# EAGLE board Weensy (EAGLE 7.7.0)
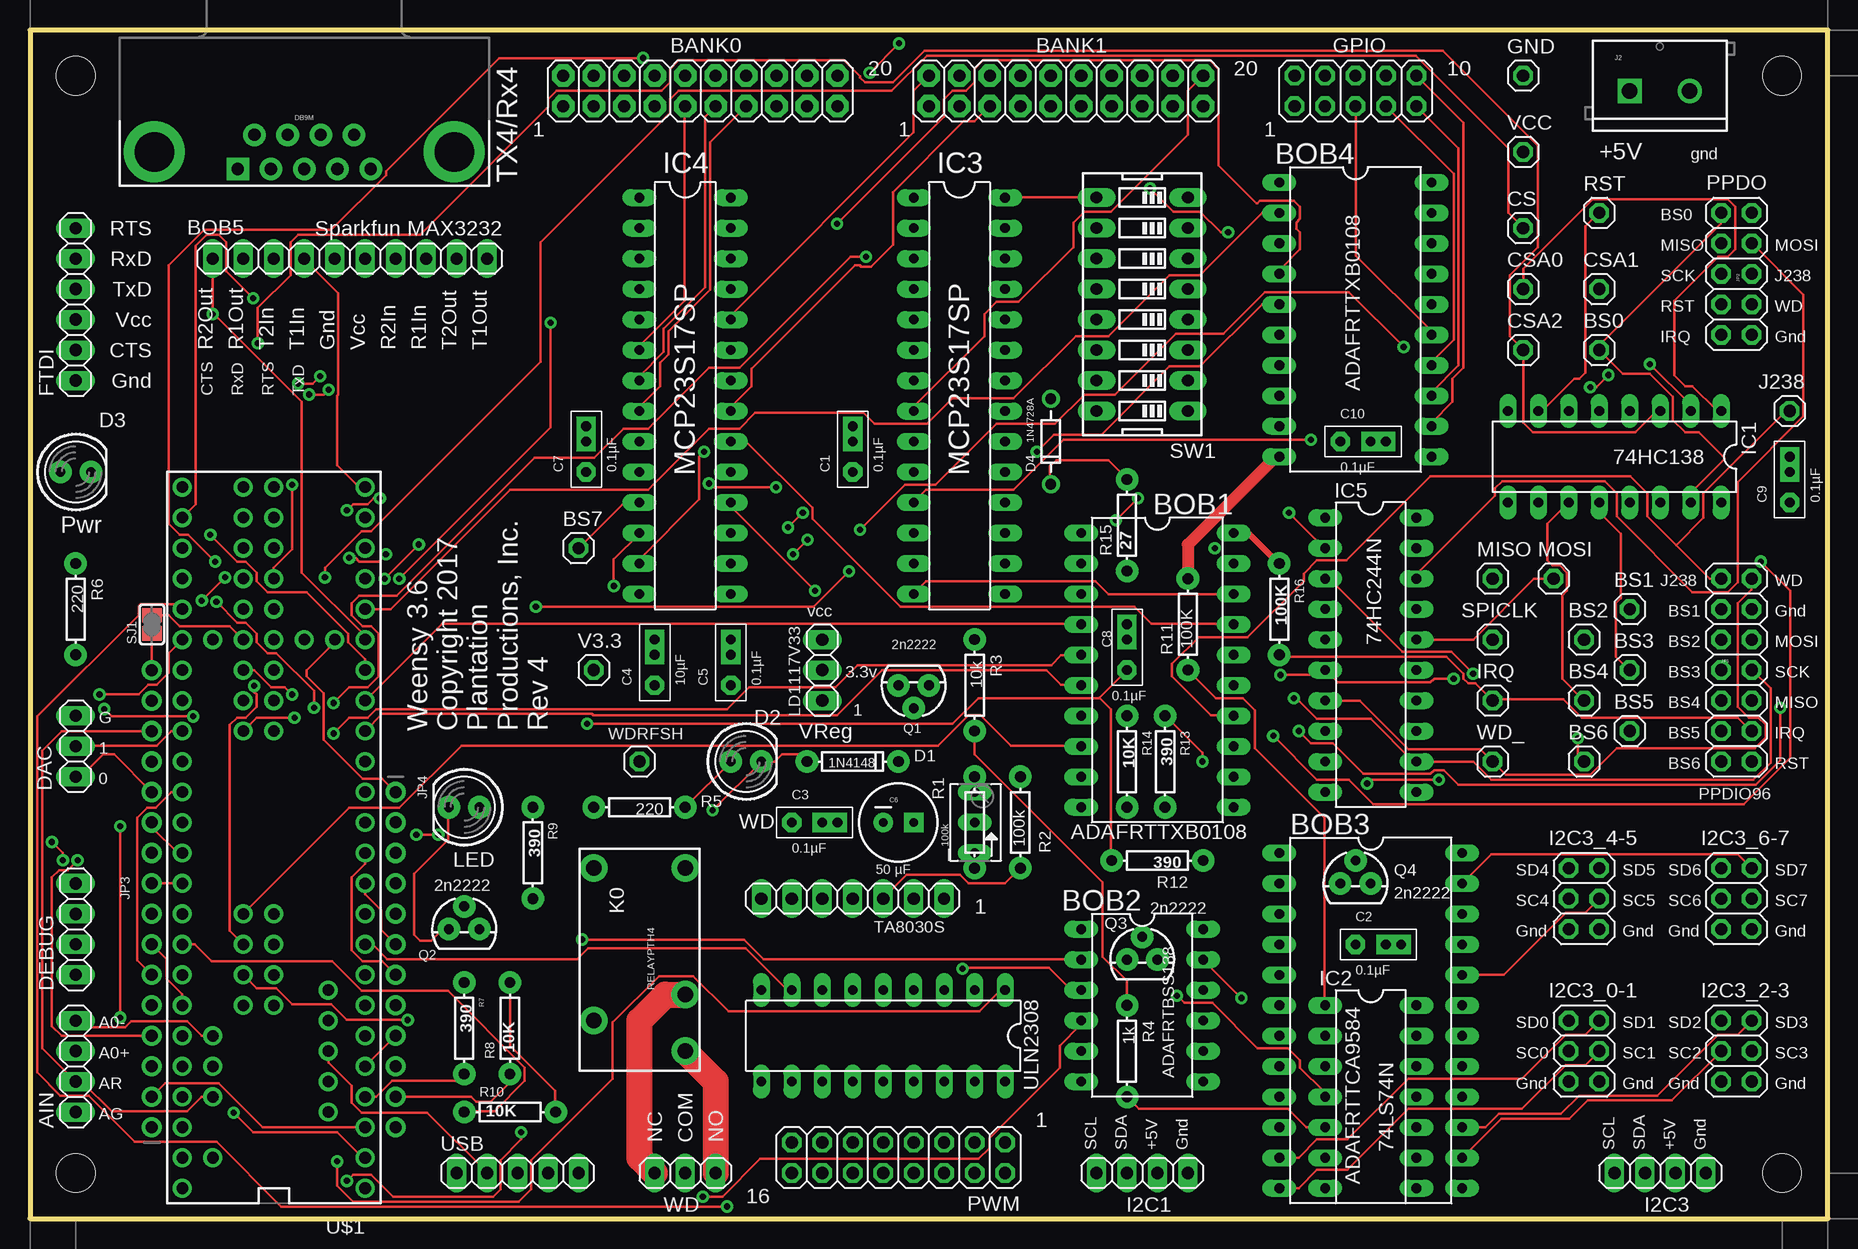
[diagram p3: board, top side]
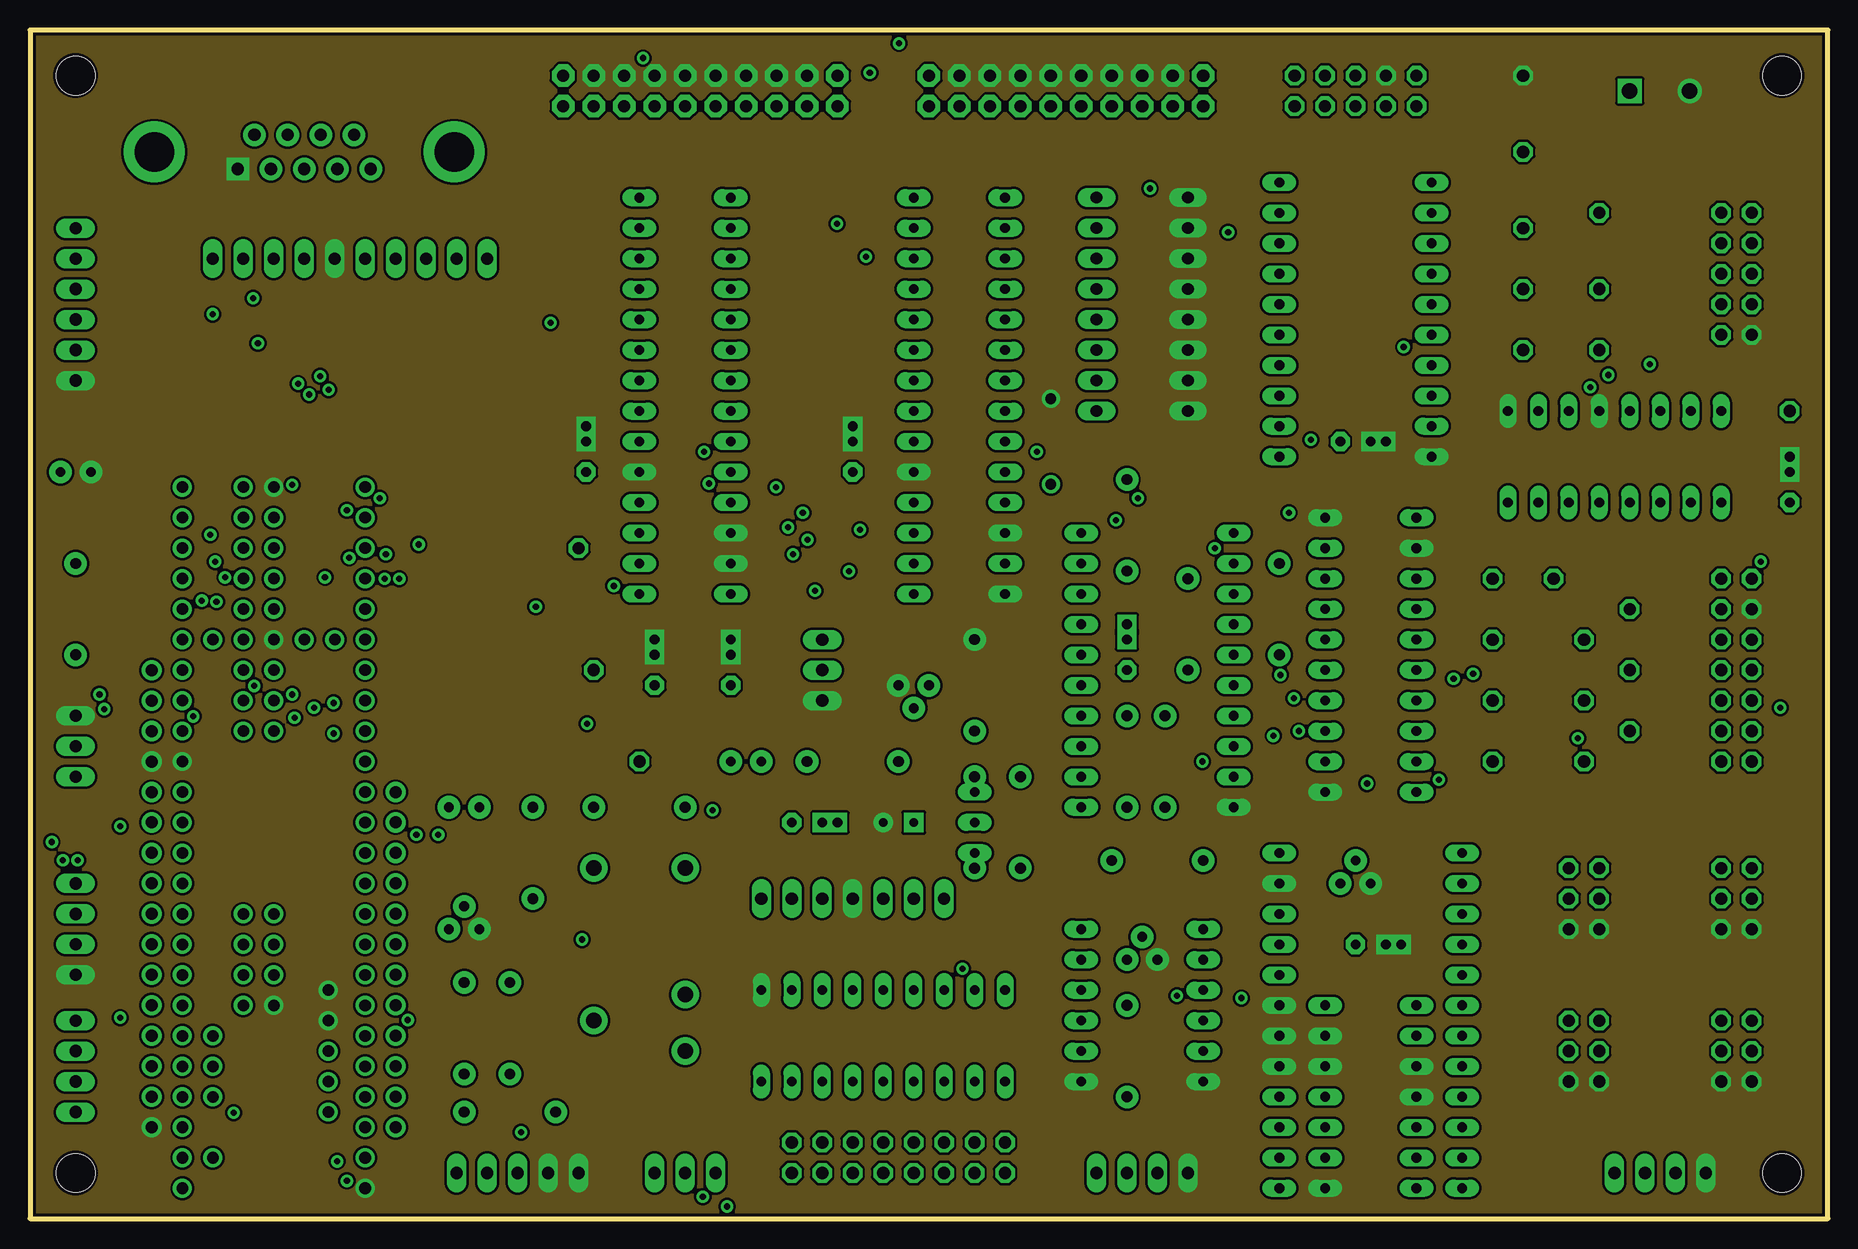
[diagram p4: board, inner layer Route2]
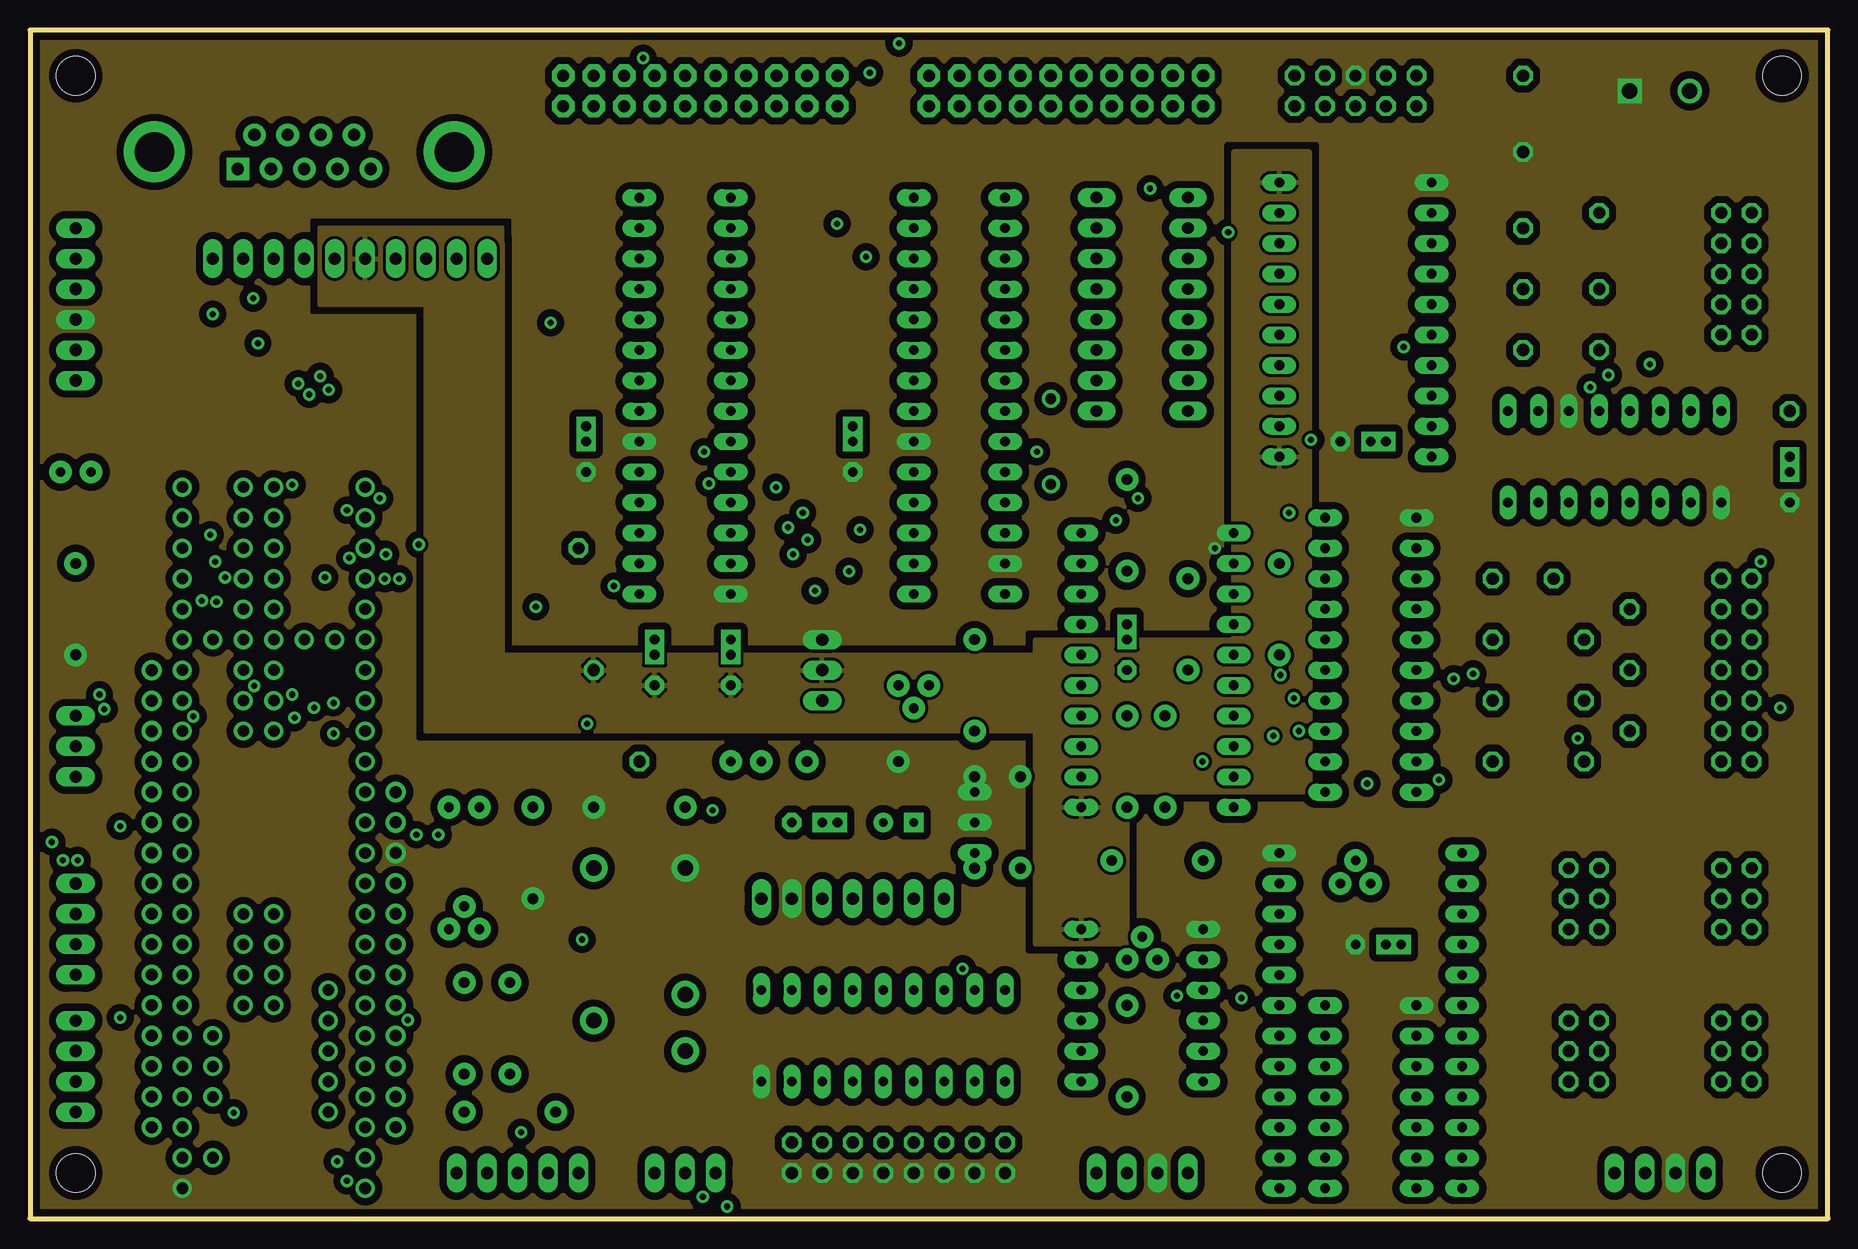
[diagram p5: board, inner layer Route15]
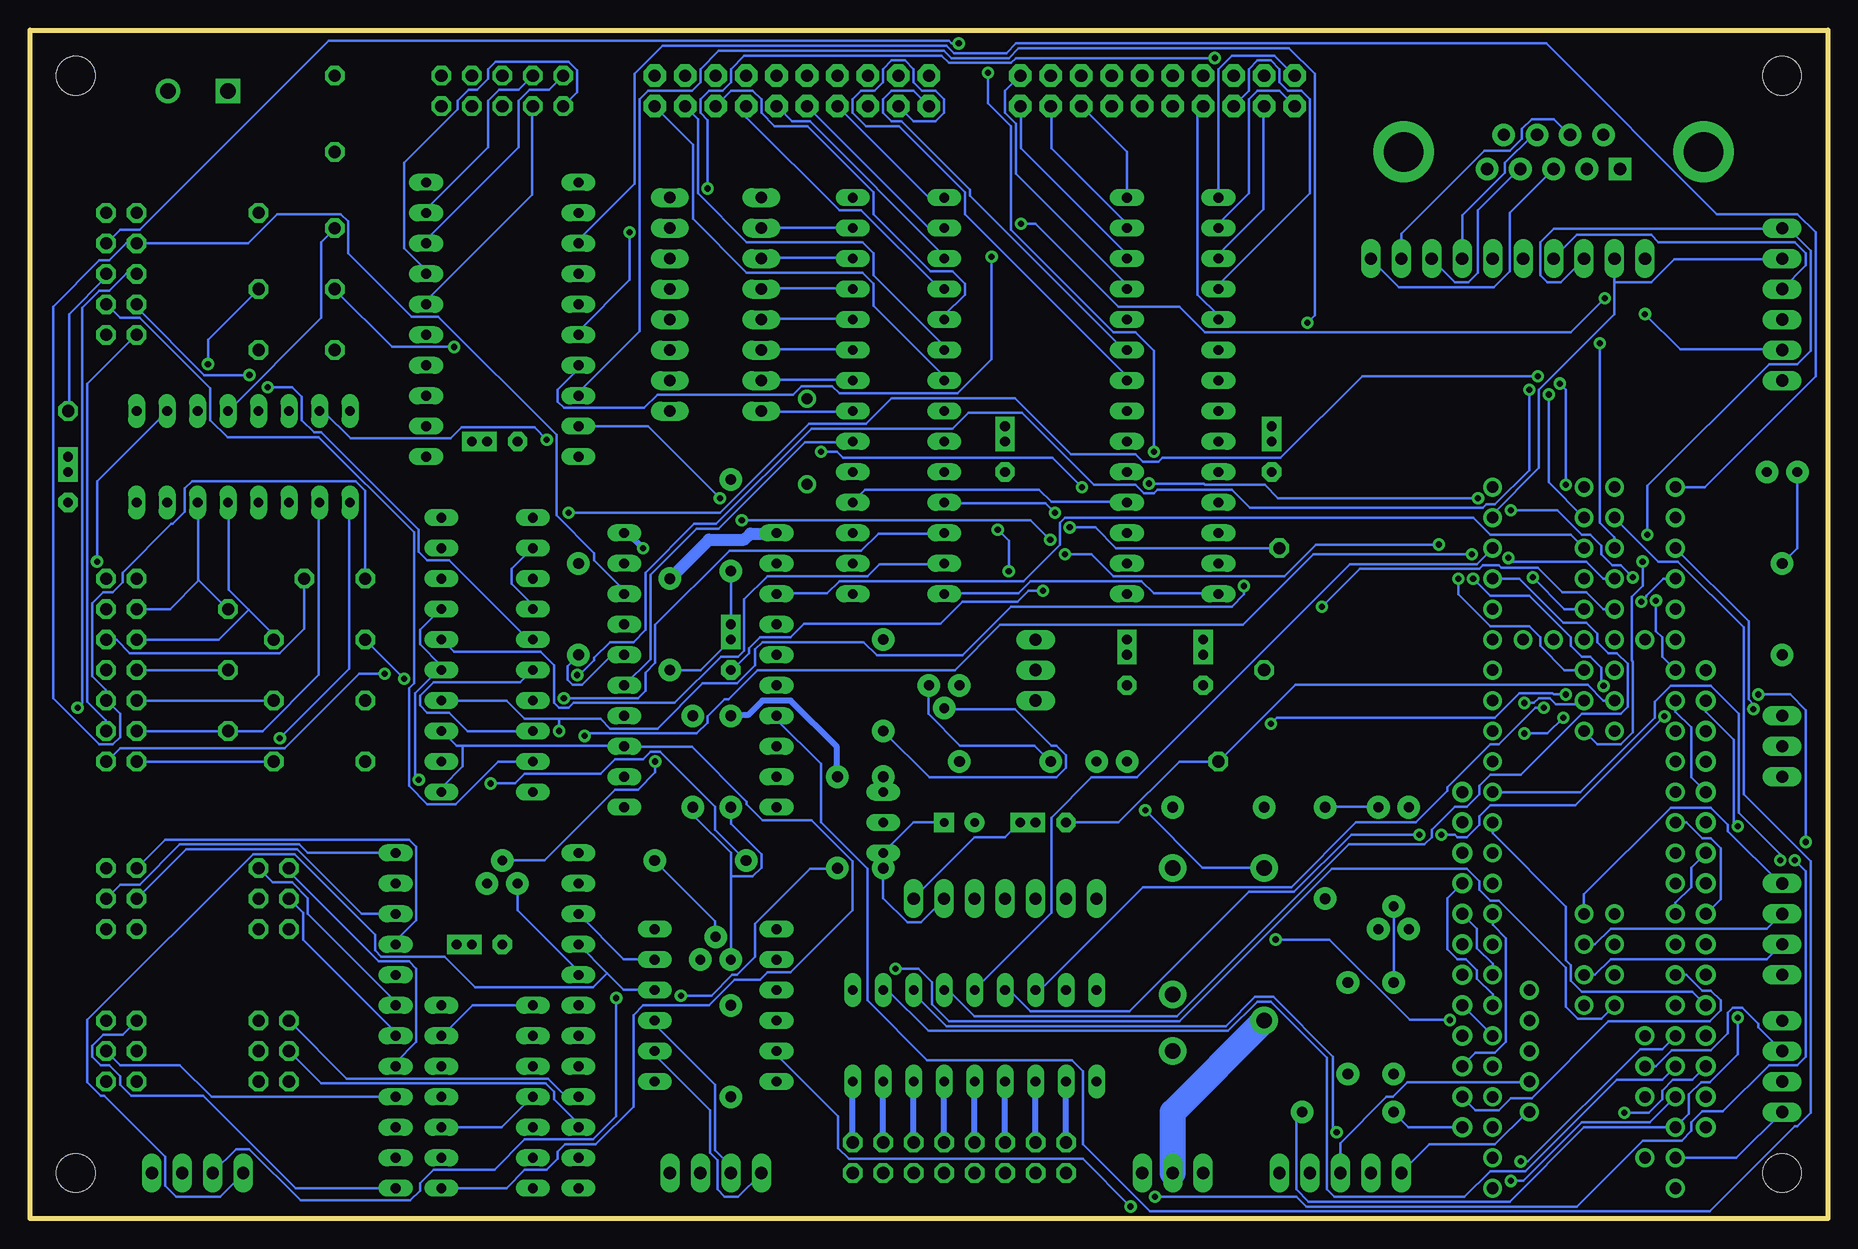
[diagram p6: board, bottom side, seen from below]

Size 149.86 x 99.06 mm. Coordinates in mm from the lower left corner, seen from the top.
Outline: 0,0 149.86,0 149.86,99.06 0,99.06 0,0
Copper layers (1*2*15*16): Top 0.035mm / dielectric 1.5mm / Route2 0.035mm / dielectric 0.15mm / Route15 0.035mm / dielectric 0.2mm / Bottom 0.035mm
Design rules "SparkFun *": minimum track width 8mil, minimum drill 20mil, track to track 8mil, track to pad 8mil, pad to pad 8mil, via to via 8mil, smd to smd 8mil, copper to edge 10mil, drill to drill 8mil, minimum pad ring 12mil, minimum via ring 10mil, stop-mask expansion 4mil, vias tented up to drill 25mil, thermal gap 10mil
Net classes: 1 Power: width 1.016 mm, drill 0.127 mm, clearance 0.254 mm; 2 Hi Current: width 0.508 mm, drill 0.254 mm, clearance 0.254 mm; 3 Relay: width 2.54 mm, drill 0.254 mm, clearance 0.254 mm
Holes 3.2 mm at 3.81,95.25 3.81,3.81 146.05,95.25 146.05,3.81

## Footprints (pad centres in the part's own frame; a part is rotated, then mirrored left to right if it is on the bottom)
B64Y = drill 0.813 long: A 2.54,0; E -2.54,0; S 0,0
1X04 = drill 1.016 long: 1 -3.81,0; 2 -1.27,0; 3 1.27,0; 4 3.81,0
2X10 = drill 1.016 pad 1.88 octagon: 1 -11.43,-1.27; 2 -11.43,1.27; 3 -8.89,-1.27; 4 -8.89,1.27; 5 -6.35,-1.27; 6 -6.35,1.27; 7 -3.81,-1.27; 8 -3.81,1.27; 9 -1.27,-1.27; 10 -1.27,1.27; 11 1.27,-1.27; 12 1.27,1.27; 13 3.81,-1.27; 14 3.81,1.27; 15 6.35,-1.27; 16 6.35,1.27; 17 8.89,-1.27; 18 8.89,1.27; 19 11.43,-1.27; 20 11.43,1.27
DIL20W = drill 0.813 long: 1 -11.43,-6.35; 2 -8.89,-6.35; 3 -6.35,-6.35; 4 -3.81,-6.35; 5 -1.27,-6.35; 6 1.27,-6.35; 7 3.81,-6.35; 8 6.35,-6.35; 9 8.89,-6.35; 10 11.43,-6.35; 11 11.43,6.35; 12 8.89,6.35; 13 6.35,6.35; 14 3.81,6.35; 15 1.27,6.35; 16 -1.27,6.35; 17 -3.81,6.35; 18 -6.35,6.35; 19 -8.89,6.35; 20 -11.43,6.35
DIL12W = drill 0.813 long: 1 -12.7,-5.08; 2 -10.16,-5.08; 3 -7.62,-5.08; 4 -5.08,-5.08; 5 -2.54,-5.08; 6 0,-5.08; 7 0,5.08; 8 -2.54,5.08; 9 -5.08,5.08; 10 -7.62,5.08; 11 -10.16,5.08; 12 -12.7,5.08
DIL24W = drill 0.813 long: 1 -13.97,-7.62; 2 -11.43,-7.62; 3 -8.89,-7.62; 4 -6.35,-7.62; 5 -3.81,-7.62; 6 -1.27,-7.62; 7 1.27,-7.62; 8 3.81,-7.62; 9 6.35,-7.62; 10 8.89,-7.62; 11 11.43,-7.62; 12 13.97,-7.62; 13 13.97,7.62; 14 11.43,7.62; 15 8.89,7.62; 16 6.35,7.62; 17 3.81,7.62; 18 1.27,7.62; 19 -1.27,7.62; 20 -3.81,7.62; 21 -6.35,7.62; 22 -8.89,7.62; 23 -11.43,7.62; 24 -13.97,7.62
1X10 = drill 1.016 long: 1 -11.43,0; 2 -8.89,0; 3 -6.35,0; 4 -3.81,0; 5 -1.27,0; 6 1.27,0; 7 3.81,0; 8 6.35,0; 9 8.89,0; 10 11.43,0
1X01 = drill 1.016 octagon: 1 0,0
1+2CAP = drill 0.813 pad 1.6 octagon: 1 -2.54,0 | drill 0.813 pad 1.6 square: 2@1 0,0; 2@2 1.27,0
CPOL-RADIAL-100UF-25V = drill 0.7 pad 1.651 square: 1 1.27,0 | drill 0.7 pad 1.651: 2 -1.27,0
DIODE-1N4148 = drill 0.9 pad 1.88: A -3.81,0; C 3.81,0
LED5MM = drill 0.813 pad 1.88: A -1.27,0; K 1.27,0
DIODE-ZENER = drill 0.9: P$1 -3.556,0; P$2 3.556,0
1X03 = drill 1.016 long: 1 -2.54,0; 2 0,0; 3 2.54,0
DB9_MALE = drill 1.016 pad 1.88: 1 5.54,-1.42; 2 2.77,-1.42; 3 0,-1.42; 4 -2.77,-1.42; 6 4.15,1.42; 7 1.38,1.42; 8 -1.38,1.42; 9 -4.15,1.42 | drill 1.016 pad 1.88 square: 5 -5.54,-1.42 | drill 3.302 pad 5.08: G1 -12.5,0; G2 12.5,0
1X06 = drill 1.016 long: 1 -6.35,0; 2 -3.81,0; 3 -1.27,0; 4 1.27,0; 5 3.81,0; 6 6.35,0
2X05 = drill 1.016 octagon: 1 -5.08,-1.27; 2 -5.08,1.27; 3 -2.54,-1.27; 4 -2.54,1.27; 5 0,-1.27; 6 0,1.27; 7 2.54,-1.27; 8 2.54,1.27; 9 5.08,-1.27; 10 5.08,1.27
2X03 = drill 1.016 octagon: 1 -2.54,-1.27; 2 -2.54,1.27; 3 0,-1.27; 4 0,1.27; 5 2.54,-1.27; 6 2.54,1.27
DIL16 = drill 0.813 long: 1 -8.89,-3.81; 2 -6.35,-3.81; 3 -3.81,-3.81; 4 -1.27,-3.81; 5 1.27,-3.81; 6 3.81,-3.81; 7 6.35,-3.81; 8 8.89,-3.81; 9 8.89,3.81; 10 6.35,3.81; 11 3.81,3.81; 12 1.27,3.81; 13 -1.27,3.81; 14 -3.81,3.81; 15 -6.35,3.81; 16 -8.89,3.81
DIL14 = drill 0.813 long: 1 -7.62,-3.81; 2 -5.08,-3.81; 3 -2.54,-3.81; 4 0,-3.81; 5 2.54,-3.81; 6 5.08,-3.81; 7 7.62,-3.81; 8 7.62,3.81; 9 5.08,3.81; 10 2.54,3.81; 11 0,3.81; 12 -2.54,3.81; 13 -5.08,3.81; 14 -7.62,3.81
DIL28-3 = drill 0.813 long: 1 -16.51,-3.81; 2 -13.97,-3.81; 3 -11.43,-3.81; 4 -8.89,-3.81; 5 -6.35,-3.81; 6 -3.81,-3.81; 7 -1.27,-3.81; 8 1.27,-3.81; 9 3.81,-3.81; 10 6.35,-3.81; 11 8.89,-3.81; 12 11.43,-3.81; 13 13.97,-3.81; 14 16.51,-3.81; 15 16.51,3.81; 16 13.97,3.81; 17 11.43,3.81; 18 8.89,3.81; 19 6.35,3.81; 20 3.81,3.81; 21 1.27,3.81; 22 -1.27,3.81; 23 -3.81,3.81; 24 -6.35,3.81; 25 -8.89,3.81; 26 -11.43,3.81; 27 -13.97,3.81; 28 -16.51,3.81
DIL20 = drill 0.813 long: 1 -11.43,-3.81; 2 -8.89,-3.81; 3 -6.35,-3.81; 4 -3.81,-3.81; 5 -1.27,-3.81; 6 1.27,-3.81; 7 3.81,-3.81; 8 6.35,-3.81; 9 8.89,-3.81; 10 11.43,-3.81; 11 11.43,3.81; 12 8.89,3.81; 13 6.35,3.81; 14 3.81,3.81; 15 1.27,3.81; 16 -1.27,3.81; 17 -3.81,3.81; 18 -6.35,3.81; 19 -8.89,3.81; 20 -11.43,3.81
SCREWTERMINAL-5MM-2 = drill 1.3 pad 2.032 square: 1 0,0 | drill 1.3 pad 2.032: 2 5,0
2X07 = drill 1.016 octagon: 1 -7.62,-1.27; 2 -7.62,1.27; 3 -5.08,-1.27; 4 -5.08,1.27; 5 -2.54,-1.27; 6 -2.54,1.27; 7 0,-1.27; 8 0,1.27; 9 2.54,-1.27; 10 2.54,1.27; 11 5.08,-1.27; 12 5.08,1.27; 13 7.62,-1.27; 14 7.62,1.27
1X16_ROUND = drill 1 pad 1.676: 1 -19.05,0; 2 -16.51,0; 3 -13.97,0; 4 -11.43,0; 5 -8.89,0; 6 -6.35,0; 7 -3.81,0; 8 -1.27,0; 9 1.27,0; 10 3.81,0; 11 6.35,0; 12 8.89,0; 13 11.43,0; 14 13.97,0; 15 16.51,0; 16 19.05,0
1X12_ROUND = drill 1 pad 1.676: 1 -13.97,0; 2 -11.43,0; 3 -8.89,0; 4 -6.35,0; 5 -3.81,0; 6 -1.27,0; 7 1.27,0; 8 3.81,0; 9 6.35,0; 10 8.89,0; 11 11.43,0; 12 13.97,0
RELAY-JZC = drill 1.3 pad 2.286: 1 3.81,-8.89; 2 -3.81,1.651; 3 -3.81,6.35; 4 3.81,3.81; 5 -3.81,-8.89
2X08 = drill 1.016 octagon: 1 -8.89,-1.27; 2 -8.89,1.27; 3 -6.35,-1.27; 4 -6.35,1.27; 5 -3.81,-1.27; 6 -3.81,1.27; 7 -1.27,-1.27; 8 -1.27,1.27; 9 1.27,-1.27; 10 1.27,1.27; 11 3.81,-1.27; 12 3.81,1.27; 13 6.35,-1.27; 14 6.35,1.27; 15 8.89,-1.27; 16 8.89,1.27
TO-92 = drill 0.813 pad 1.88: 1 -1.27,0; 2 0,1.905; 3 1.27,0
AXIAL-0.3 = drill 0.9 pad 1.88: P$1 -3.81,0; P$2 3.81,0
SOLDERJUMPER_CLOSEDWIRE = smd 1.168 x 1.6: 1 -0.762,0; 2 0.762,0 | smd 0.635 x 0.203: WIRE 0,0
DIPSWITCH-08 = drill 0.97 long: 1 -8.89,-3.81; 2 -6.35,-3.81; 3 -3.81,-3.81; 4 -1.27,-3.81; 5 1.27,-3.81; 6 3.81,-3.81; 7 6.35,-3.81; 8 8.89,-3.81; 9 8.89,3.81; 10 6.35,3.81; 11 3.81,3.81; 12 1.27,3.81; 13 -1.27,3.81; 14 -3.81,3.81; 15 -6.35,3.81; 16 -8.89,3.81
1X07 = drill 1.016 long: 1 -7.62,0; 2 -5.08,0; 3 -2.54,0; 4 0,0; 5 2.54,0; 6 5.08,0; 7 7.62,0
TEENSY-3.6_FULL = drill 0.965: 0 -7.62,5.08; 1 -7.62,2.54; 2 -7.62,0; 3 -7.62,-2.54; 3.3V_2 -2.54,-38.1; 3V3_1 -7.62,-27.94; 3V3_3 2.54,-50.8; 3V3_MAX_250 7.62,2.54; 4 -7.62,-5.08; 5 -7.62,-7.62; 6 -7.62,-10.16; 7 -7.62,-12.7; 8 -7.62,-15.24; 9 -7.62,-17.78; 10 -7.62,-20.32; 11 -7.62,-22.86; 12 -7.62,-25.4; 13 7.62,-25.4; 14 7.62,-22.86; 15 7.62,-20.32; 16 7.62,-17.78; 17 7.62,-15.24; 18 7.62,-12.7; 19 7.62,-10.16; 20 7.62,-7.62; 21 7.62,-5.08; 22 7.62,-2.54; 23 7.62,0; 24 -7.62,-30.48; 25 -7.62,-33.02; 26 -7.62,-35.56; 27 -7.62,-38.1; 28 -7.62,-40.64; 29 -7.62,-43.18; 30 -7.62,-45.72; 31 -7.62,-48.26; 32 -7.62,-50.8; 33 7.62,-50.8; 34 7.62,-48.26; 35 7.62,-45.72; 36 7.62,-43.18; 37 7.62,-40.64; 38 7.62,-38.1; 39 7.62,-35.56; 40 0,-30.48; 41 0,-33.02; 42 0,-35.56; 43 0,-40.64; 44 0,-43.18; 45 0,-45.72; 46 0,-48.26; 47 2.54,-48.26; 48 2.54,-45.72; 49 2.54,-43.18; 50 2.54,-40.64; 51 2.54,-35.56; 52 2.54,-33.02; 53 2.54,-30.48; 54 2.54,-15.24; 55 2.54,-12.7; 56 2.54,-10.16; 57 2.54,-7.62; +5V -4.547,1.27; A10 5.08,-2.54; A11 5.08,-5.08; A21 7.62,-33.02; A22 7.62,-30.48; AGND 7.62,5.08; AREF 5.08,0; D+ -4.547,-3.81; D- -4.547,-1.27; DC 0,-12.7; DD 0,-15.24; DE 0,-10.16; GND1 -7.62,7.62; GND2 7.62,-27.94; GND3 -4.547,-6.35; GND4 -4.547,-8.89; GND5 0,-38.1; GND6 0,-7.62; GND7 0,-50.8; PROGRAM 2.54,-38.1; RESET 5.08,-38.1; VBAT -5.08,-38.1; VIN 7.62,7.62; VUSB 5.08,5.08
DIL18 = drill 0.813 long: 1 -10.16,-3.81; 2 -7.62,-3.81; 3 -5.08,-3.81; 4 -2.54,-3.81; 5 0,-3.81; 6 2.54,-3.81; 7 5.08,-3.81; 8 7.62,-3.81; 9 10.16,-3.81; 10 10.16,3.81; 11 7.62,3.81; 12 5.08,3.81; 13 2.54,3.81; 14 0,3.81; 15 -2.54,3.81; 16 -5.08,3.81; 17 -7.62,3.81; 18 -10.16,3.81
1X05 = drill 1.016 long: 1 -5.08,0; 2 -2.54,0; 3 0,0; 4 2.54,0; 5 5.08,0

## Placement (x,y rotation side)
_  [B64Y]  78.74,33.02 90 top
AIN  [1X04]  3.81,12.7 90 top
BANK0  [2X10]  55.88,93.98 0 top
BANK1  [2X10]  86.36,93.98 0 top
BOB1  ADAFRTTXB0108  [DIL20W]  93.98,45.72 270 top
BOB2  ADAFRTBSS138  [DIL12W]  92.71,11.43 270 top
BOB3  ADAFRTTCA9584  [DIL24W]  111.76,16.51 270 top
BOB4  ADAFRTTXB0108  [DIL20W]  110.49,74.93 270 top
BOB5  Sparkfun MAX3232  [1X10]  26.67,80.01 180 top
BS0  [1X01]  130.81,72.39 0 top
BS1  [1X01]  133.35,50.8 0 top
BS2  [1X01]  129.54,48.26 0 top
BS3  [1X01]  133.35,45.72 0 top
BS4  [1X01]  129.54,43.18 0 top
BS5  [1X01]  133.35,40.64 0 top
BS6  [1X01]  129.54,38.1 0 top
BS7  [1X01]  45.72,55.88 0 top
C1  0.1µF  [1+2CAP]  68.58,64.77 90 top
C2  0.1µF  [1+2CAP]  113.03,22.86 0 top
C3  0.1µF  [1+2CAP]  66.04,33.02 0 top
C4  10µF  [1+2CAP]  52.07,46.99 90 top
C5  0.1µF  [1+2CAP]  58.42,46.99 90 top
C6  50 µF  [CPOL-RADIAL-100UF-25V]  72.39,33.02 0 top
C7  0.1µF  [1+2CAP]  46.35,64.77 90 top
C8  0.1µF  [1+2CAP]  91.44,48.26 90 top
C9  0.1µF  [1+2CAP]  146.69,62.23 90 top
C10  0.1µF  [1+2CAP]  111.76,64.77 0 top
CS  [1X01]  124.46,82.55 0 top
CSA0  [1X01]  124.46,77.47 0 top
CSA1  [1X01]  130.81,77.47 0 top
CSA2  [1X01]  124.46,72.39 0 top
D1  1N4148  [DIODE-1N4148]  68.58,38.1 0 top
D2  WD  [LED5MM]  59.69,38.1 0 top
D3  [LED5MM]  3.81,62.23 0 top
D4  1N4728A  [DIODE-ZENER]  85.09,64.77 90 top
DAC  [1X03]  3.81,39.37 270 top
DB9M  [DB9_MALE]  22.86,88.9 0 top
DEBUG  [1X04]  3.81,24.13 90 top
FRAME1  FRAME-LETTERNO_PACKAGE  [DUMMY]  0,1.27 0 top
FRAME2  FRAME-LETTERNO_PACKAGE  [DUMMY]  120.65,5.08 0 top
FRAME3  FRAME-LETTER  [CREATIVE_COMMONS]  not placed on the board
FTDI  [1X06]  3.81,76.2 90 top
GND  [1X01]  124.46,95.25 0 top
GPIO  [2X05]  110.49,93.98 0 top
I2C1  [1X04]  92.71,3.81 0 top
I2C3  [1X04]  135.89,3.81 0 top
I2C3_0-1  [2X03]  129.54,13.97 270 top
I2C3_2-3  [2X03]  142.24,13.97 270 top
I2C3_4-5  [2X03]  129.54,26.67 270 top
I2C3_6-7  [2X03]  142.24,26.67 270 top
IC1  74HC138  [DIL16]  132.08,63.5 180 top
IC2  74LS74N  [DIL14]  111.76,10.16 270 top
IC3  MCP23S17SP  [DIL28-3]  77.47,68.58 270 top
IC4  MCP23S17SP  [DIL28-3]  54.61,68.58 270 top
IC5  74HC244N  [DIL20]  111.76,46.99 270 top
IRQ  [1X01]  121.92,43.18 0 top
J2  [SCREWTERMINAL-5MM-2]  133.35,93.98 0 top
J238  [1X01]  146.69,67.31 0 top
JP1  PPDIO96  [2X07]  142.24,45.72 270 top
JP2  PPDO  [2X05]  142.24,78.74 270 top
JP3  [1X16_ROUND]  10.16,26.67 90 top
JP4  [1X12_ROUND]  30.48,21.59 270 top
K0  RELAYPTH4  [RELAY-JZC]  50.8,20.32 180 top
LD1117V33  VReg  [1X03]  66.04,45.72 90 top
LED  [LED5MM]  36.2,34.29 180 top
MISO  [1X01]  121.92,53.34 0 top
MOSI  [1X01]  127,53.34 0 top
PWM  [2X08]  72.39,5.08 180 top
Q1  2n2222  [TO-92]  73.66,44.45 180 top
Q2  2n2222  [TO-92]  36.2,24.13 0 top
Q3  2n2222  [TO-92]  92.71,21.59 0 top
Q4  2n2222  [TO-92]  110.49,27.94 0 top
R1  100k  [AXIAL-0.3]  78.74,33.02 90 top
R2  100k  [AXIAL-0.3]  82.55,33.02 90 top
R3  10k  [AXIAL-0.3]  78.74,44.45 270 top
R4  1k  [AXIAL-0.3]  91.44,13.97 270 top
R5  220  [AXIAL-0.3]  50.8,34.29 180 top
R6  220  [AXIAL-0.3]  3.81,50.8 270 top
R7  390  [AXIAL-0.3]  36.2,15.88 270 top
R8  10K  [AXIAL-0.3]  40.01,15.88 90 top
R9  390  [AXIAL-0.3]  41.91,30.48 270 top
R10  10K  [AXIAL-0.3]  40.01,8.89 0 top
R11  100K  [AXIAL-0.3]  96.52,49.53 90 top
R12  390  [AXIAL-0.3]  93.98,29.84 180 top
R13  390  [AXIAL-0.3]  94.61,38.1 270 top
R14  10K  [AXIAL-0.3]  91.44,38.1 270 top
R15  27  [AXIAL-0.3]  91.44,57.78 90 top
R16  100K  [AXIAL-0.3]  104.14,50.8 270 top
RST  [1X01]  130.81,83.82 0 top
SJ1  [SOLDERJUMPER_CLOSEDWIRE]  10.16,49.53 90 top
SPICLK  [1X01]  121.92,48.26 0 top
SW1  [DIPSWITCH-08]  92.71,76.2 90 top
TA8030S  [1X07]  68.58,26.67 180 top
U$1  [TEENSY-3.6_FULL]  20.32,10.16 180 top
ULN2308  [DIL18]  71.12,15.24 180 top
USB  [1X05]  40.64,3.81 0 top
V3.3  [1X01]  46.99,45.72 0 top
VCC  [1X01]  124.46,88.9 0 top
WD  [1X03]  54.61,3.81 0 top
WD_  [1X01]  121.92,38.1 0 top
WDRFSH  [1X01]  50.8,38.1 0 top

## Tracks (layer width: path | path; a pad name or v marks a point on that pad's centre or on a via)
3
  Top 0.203: JP4.9 U$1.3
3V3_MAX_250  (via drill 0.51)
  Top 0.203: v7.52,16.76 v7.52,32.72 | R8.P$2 40.03,19.61 40.03,14.43 43.79,10.67 43.79,8.94 R10.P$2
  Bottom 0.203: R10.P$2 43.89,8.84 44.3,8.43 44.3,2.44 43.28,1.42 26.52,1.42 20.32,7.62 U$1.3V3_MAX_250 11.58,8.74 11.58,10.36 10.57,11.38 9.86,11.38 7.52,13.72 v7.52,16.76 | JP3.15 10.16,42.27 7.82,39.93 7.82,33.02 v7.52,32.72
4
  Bottom 0.203: JP4.8 U$1.4
5
  Bottom 0.203: U$1.5 27.94,18.69 29.26,20.02 29.26,20.73 30.18,21.64 30.89,21.64 31.7,22.45 31.7,26.72 JP4.4
6
  Bottom 0.203: U$1.6 27.94,21.23 29.26,22.55 29.26,24.18 JP4.5
8
  Bottom 0.203: U$1.8 27.94,24.49 26.82,23.37 26.82,14.73 27.74,13.82 29.36,13.82 JP4.10
9
  Top 0.203: U$1.9 27.94,27.03 29.26,25.7 29.26,24.08 JP4.6
10
  Top 0.203: U$1.10 27.94,29.57 26.82,28.45 26.82,22.35 27.74,21.44 29.36,21.44 JP4.7
24
  Top 0.203: U$1.24 29.36,42.06 46.84,42.06 46.94,41.96 67.26,41.96 71.02,45.72 84.73,45.72 85.95,44.5 87.58,44.5 BOB1.6
25
  Top 0.203: U$1.25 34.34,49.58 87.58,49.58 BOB1.4
28
  Top 0.203: BOB4.2 102.72,83.82 97.54,78.64 95,78.64 89.92,73.56 87.17,73.56 81.99,68.38 76.91,68.38 74.78,66.24 70.41,66.24 69.49,67.16 60.45,67.16 59.13,65.84 56.59,65.84 51.51,60.76 40.03,60.76 30.07,50.8 U$1.28
33
  Bottom 0.203: BOB4.3 104.14,81.58 99.47,86.26 99.47,95.4 97.13,97.74 73.46,97.74 72.85,97.13 68.48,97.13 67.67,97.94 23.47,97.94 9.25,83.72 2.54,83.72 1.02,82.19 1.02,70.21 10.26,60.96 U$1.33
34  (via drill 0.51)
  Top 0.203: BOB4.4 104.14,79.05 105.87,80.77 105.87,82.19 105.56,82.5 105.56,83.01 105.87,83.31 105.87,84.33 105.36,84.84 102.51,84.84 102.31,84.63 102.21,84.63 99.06,87.78 99.06,95.81 98.35,96.52 79.45,96.52 78.74,95.81 78.74,94.69 78.03,93.98 76.91,93.98 76.2,93.27 76.2,91.85 v67.26,82.91 | v18.59,76.71 16.36,78.94 16.36,81.38 15.75,81.99 14.73,81.99 13.82,81.08 13.82,59.54 U$1.34
  Bottom 0.203: v67.26,82.91 66.04,82.91 59.13,76 54.05,76 51.92,73.86 21.44,73.86 v18.59,76.71
39  (via drill 0.51)
  Top 0.203: BOB4.5 102.72,76.2 97.54,71.02 95,71.02 89.31,65.33 85.34,65.33 v83.92,63.91 | v62.18,60.96 56.9,60.96 v56.59,61.27 | v29.16,60.05 28.65,60.05 28.14,59.54 26.92,59.54 v26.42,59.03 | v14.33,51.51 v16.26,53.44
  Bottom 0.203: v83.92,63.91 82.6,63.91 82.09,63.4 64.62,63.4 v62.18,60.96 | v56.59,61.27 52.02,61.27 51.92,61.16 46.94,61.16 45.82,60.05 v29.16,60.05 | v26.42,59.03 22.55,59.03 20.52,57 19.81,57 18.9,56.08 18.9,55.37 17.98,54.46 17.27,54.46 v16.26,53.44 | v14.33,51.51 14.33,48.97 13.82,48.46 13.82,46.84 U$1.39
40  (via drill 0.51)
  Top 0.203: v99.87,82.19 99.26,82.19 97.54,83.92 95.3,83.92 v93.37,85.85 | v51.1,96.72 39.12,96.72 29.67,87.27 29.67,86.97 25.09,82.4 14.53,82.4 11.58,79.45 11.58,57.91 12.5,57 13.21,57 v15.44,54.76
  Bottom 0.203: BOB4.6 104.14,73.97 99.87,78.23 v99.87,82.19 | v93.37,85.85 93.37,91.54 93.98,92.15 93.98,93.27 93.27,93.98 92.15,93.98 91.44,94.69 91.44,95.81 90.32,96.93 73.86,96.93 73.25,96.32 68.07,96.32 67.67,96.72 v51.1,96.72 | v15.44,54.76 15.44,52.73 16.36,51.82 16.36,46.53 16.26,46.43 16.26,40.54 17.27,39.52 19.2,39.52 U$1.40
41  (via drill 0.51)
  Top 0.203: v69.7,80.16 68.38,80.16 59.13,70.92 56.59,70.92 51.51,65.84 49.48,65.84 47.04,63.4 42.06,63.4 30.58,51.92 27.43,51.92 26.82,51.31 26.82,50.29 27.74,49.38 28.45,49.38 29.06,48.77 29.06,45.21 28.14,44.3 26.62,44.3 v25.3,42.98
  Bottom 0.203: BOB4.7 104.14,70.81 105.87,69.09 105.87,68.07 105.36,67.56 98.65,67.56 97.54,68.68 86.26,68.68 85.55,69.39 83.01,69.39 82.4,68.78 72.54,68.78 69.7,71.63 v69.7,80.16 | v25.3,42.98 24.49,42.98 24.08,43.38 23.16,43.38 22.66,42.88 20.62,42.88 U$1.41
42  (via drill 0.51)
  Top 0.203: v43.38,74.68 43.38,65.94 v30.79,53.34
  Bottom 0.203: BOB4.8 104.14,68.89 99.06,73.97 99.06,93.27 98.35,93.98 94.69,93.98 93.98,94.69 93.98,95.81 92.46,97.33 73.66,97.33 73.05,96.72 68.28,96.72 67.46,97.54 44.91,97.54 42.77,95.4 42.77,75.29 v43.38,74.68 | v30.79,53.34 30.79,52.02 28.14,49.38 24.89,49.38 23.98,48.46 23.98,47.75 21.95,45.72 U$1.42
55  (via drill 0.51)
  Top 0.203: v90.53,58.22 v92.35,60.05 | v63.6,55.37 v64.82,56.59 | v29.57,53.34 v32.41,56.19 | v18.69,44.4 18.69,43.89 18.9,43.69 18.9,42.67 17.98,41.76 17.27,41.76 16.66,41.15 16.66,23.98 U$1.55
  Bottom 0.203: BOB4.9 98.35,66.04 v92.35,60.05 | v90.53,58.22 66.45,58.22 v64.82,56.59 | v63.6,55.37 61.37,55.37 59.54,53.54 45.31,53.54 42.67,56.19 v32.41,56.19 | v29.57,53.34 28.14,51.92 24.89,51.92 21.44,48.46 21.44,47.75 20.52,46.84 19.81,46.84 18.9,45.92 18.9,44.6 v18.69,44.4
+3V3
  Top 1.016: R11.P$2 96.52,56.19 103.83,63.5 BOB4.10
  Bottom 1.016: R11.P$2 93.27,56.59 90.32,56.59 89.81,57.1 87.68,57.1 BOB1.1
  pour Route15: 64.77,46.99 91.44,46.99 91.44,41.91 64.77,41.91
  pour Route15: 100.33,88.9 100.33,39.37 106.68,39.37 106.68,88.9
  pour Route15: 91.44,22.86 83.82,22.86 83.82,48.26 106.68,48.26 106.68,35.56 91.44,35.56
  pour Route15: 33.02,46.99 86.36,46.99 86.36,40.64 33.02,40.64
  pour Route15: 39.37,44.45 39.37,82.55 24.13,82.55 24.13,76.2 33.02,76.2 33.02,44.45
  pour Route15: 39.37,81.28 39.37,44.45 33.02,44.45 33.02,76.2
A0
  Bottom 0.203: U$1.14 11.79,33.02 10.46,31.7 9.75,31.7 8.94,30.89 8.94,26.62 JP3.8
A1
  Top 0.203: U$1.15 12.29,30.48 10.16,32.61 JP3.11
A2
  Top 0.203: JP3.9 U$1.16
A3
  Bottom 0.203: U$1.17 12.7,26.31 11.38,27.64 11.38,29.26 JP3.10
A6
  Top 0.203: U$1.20 12.7,18.69 11.38,20.02 11.38,21.64 JP3.7
ADC+
  Bottom 0.203: U$1.A10 14.33,12.7 13.01,14.02 9.75,14.02 8.33,15.44 8.33,17.17 7.92,17.58 7.11,17.58 5.79,16.26 5.79,15.95 AIN.3
ADC-
  Top 0.203: U$1.A11 14.33,15.24 13.11,16.46 8.43,16.46 7.92,15.95 4.37,15.95 AIN.4
AGND
  Bottom 0.203: U$1.AGND 7.62,5.08 AIN.1
AREF
  Top 0.203: U$1.AREF 14.33,10.16 13.11,8.94 6.81,8.94 4.37,11.38 3.86,11.38 AIN.2 1.02,14.22 1.02,39.01 2.64,40.64 JP3.14
BS0
  Top 0.203: IC1.15 138.48,59.74 138.48,60.55 141.22,63.3 141.22,63.4 139.09,65.53 137.97,65.53 136.96,66.55 136.96,68.48 135.03,70.41 132.79,70.41 BS0.1 130.86,72.44 130.86,72.85 140.92,82.91 140.92,83.82 JP2.1
BS1
  Bottom 0.203: 135.79,53.19 133.4,50.8 BS1.1 | 135.79,53.19 135.84,53.24 135.84,59.64 IC1.14 | JP1.3 138.18,50.8 135.79,53.19
BS2
  Bottom 0.203: 131.62,50.75 129.54,48.67 BS2.1 | 131.62,50.75 133.3,52.43 133.3,59.64 IC1.13 | JP1.5 134.11,48.26 131.62,50.75
BS3
  Top 0.203: IC1.12 130.86,59.64 130.86,58.83 132.59,57.1 132.59,51.71 132.18,51.31 132.18,46.84 133.3,45.72 BS3.1
  Bottom 0.203: BS3.1 JP1.7
BS4
  Top 0.203: IC1.11 126.49,57.91 126.49,54.86 126.9,54.46 127.51,54.46 128.12,53.85 128.12,52.32 127.71,51.92 127.71,45.01 BS4.1
  Bottom 0.203: BS4.1 JP1.9
BS5
  Bottom 0.203: IC1.10 125.78,59.64 125.78,45.31 130.45,40.64 BS5.1 JP1.11
BS6  (via drill 0.51)
  Top 0.203: v129.03,40.03 129.03,38.61 BS6.1
  Bottom 0.203: v129.03,40.03 123.24,45.82 123.24,59.64 IC1.9 | BS6.1 JP1.13
BS7  (via drill 0.51)
  Top 0.203: IC1.7 125.78,67.36 126.09,67.36 128.73,70 129.13,70 129.64,70.51 129.64,82.7 130.76,83.82 RST.1 | BS7.1 49.48,59.64 50.8,59.64 IC4.11 | v63.2,57.61 v64.41,58.83 | v106.78,64.92 86.16,64.92 81.99,60.76 74.68,60.76 73.66,59.74 IC3.11
  Bottom 0.203: v64.41,58.83 65.23,59.64 73.66,59.64 IC3.11 | v63.2,57.61 61.06,57.61 59.33,55.88 BS7.1 | v106.78,64.92 107.8,65.94 113.89,65.94 114.81,65.02 123.14,65.02 125.37,67.26 125.68,67.26 IC1.7
CS2  (via drill 0.51)
  Top 0.203: v24.59,53.44 24.59,54.25 27.64,57.3 28.45,57.3 42.57,71.42 42.57,81.38 53.34,92.15 53.34,93.27 54.05,93.98 71.83,93.98 74.78,96.93 115.52,96.93 123.24,89.2 123.24,83.82 124.46,82.6 CS.1
  Bottom 0.203: IC1.4 125.58,75.08 125.58,81.38 124.46,82.5 CS.1 | U$1.43 21.95,50.8 v24.59,53.44
CSA0  (via drill 0.51)
  Top 0.203: CSA0.1 124.46,79.15 130.25,84.94 141.53,84.94 142.14,84.33 142.14,80.77 141.53,80.16 140.72,80.16 137.06,76.5 137.06,70.31 137.97,69.39 138.58,69.39 140.61,67.36 140.92,67.36 IC1.1 | v42.16,51 65.33,51 v68.28,53.95 | v69.19,57.4 72.95,61.16 75.49,61.16 80.57,66.24 85.45,66.24 87.88,68.68 90.42,68.68 95.5,73.76 99.47,73.76 102.92,77.22 109.93,77.22 v114.5,72.64
  Bottom 0.203: U$1.50 18.69,50.8 20.12,52.22 22.15,52.22 24.18,54.25 27.23,54.25 27.43,54.46 28.75,54.46 29.06,54.15 39.01,54.15 v42.16,51 | v68.28,53.95 68.28,56.49 v69.19,57.4 | v114.5,72.64 119.69,72.64 124.46,77.42 CSA0.1
CSA1  (via drill 0.51)
  Top 0.203: v135.03,71.22 138.38,67.87 138.38,67.36 IC1.2 | v26.62,55.07 27.13,55.07 27.43,54.76 29.06,54.76 v29.67,55.37 | v103.63,40.23 107.29,36.58 109.93,36.58 111.96,34.54 142.85,34.54 146.71,38.41 146.71,52.32 v144.27,54.76
  Bottom 0.203: v135.03,71.22 135.03,73.25 CSA1.1 | U$1.49 18.69,53.34 20.12,54.76 26.31,54.76 v26.62,55.07 | v29.67,55.37 42.88,55.37 48.77,49.48 68.99,49.48 72.75,45.72 89.2,45.72 91.64,43.28 91.95,43.28 93.37,41.86 93.37,41.35 94.28,40.44 103.43,40.44 v103.63,40.23 | v144.27,54.76 144.27,61.47 IC1.2
CSA2  (via drill 0.51)
  Top 0.203: IC1.3 135.84,67.26 135.53,67.26 133.81,65.53 125.27,65.53 124.46,66.34 CSA2.1 124.46,72.44 123.34,73.56 123.34,78.64 125.68,80.97 125.68,89.41 117.75,97.33 74.57,97.33 71.93,94.69 69.6,94.69 69.19,95.1 69.19,95.2 67.87,96.52 54.05,96.52 53.34,95.81 53.34,94.69 52.63,93.98 43.89,93.98 43.18,93.27 43.18,92.66 32.51,81.99 22.35,81.99 21.74,81.38 21.74,78.64 19,75.89 v19,72.95
  Bottom 0.203: U$1.48 17.78,56.79 19,58.01 v19,72.95
CTS4  (via drill 0.51)
  Top 0.203: U$1.27 27.94,48.56 22.66,53.85 22.66,68.07 15.29,75.44 | 15.29,75.44 15.24,75.49 BOB5.10 | v15.24,75.39 15.29,75.44
  Bottom 0.203: v15.24,75.39 12.29,72.44 3.86,72.44 FTDI.2
DAC0
  Top 0.203: JP3.12 7.01,38.71 6.1,38.71 4.27,36.88 3.86,36.88 DAC.3
  Bottom 0.203: U$1.A21 12.7,42.27 11.38,40.95 11.38,36.78 JP3.12
DAC1
  Top 0.203: U$1.A22 11.79,40.64 10.57,39.42 3.86,39.42 DAC.2
DI_RESET  (via drill 0.51)
  Top 0.203: IC5.3 108.31,53.34 114.4,47.24 118.47,47.24 v120.29,45.41
  Bottom 0.203: v120.29,45.41 122.43,45.41 128.63,39.22 142.34,39.22 143.46,38.1 JP1.14
DI_WD_LATCH
  Top 0.203: IC5.7 110.85,43.18 114.91,39.12 120.9,39.12 WD_.1 123.04,36.98 130.05,36.98 132.28,39.22 143.76,39.22 144.68,40.13 144.68,41.15 144.07,41.76 143.26,41.76 142.34,42.67 142.34,51.31 143.46,52.43 143.46,53.34 JP1.2
DIMOSI
  Top 0.203: IC5.16 120.29,48.26 125.37,53.34 MOSI.1
  Bottom 0.203: IC3.13 73.66,54.56 79.05,54.56 80.06,53.54 88.39,53.54 90.32,51.61 90.32,47.35 90.83,46.84 92.25,46.84 96.11,42.98 104.55,42.98 104.95,42.57 105.77,42.57 106.17,42.98 106.17,46.13 107.29,47.24 114.5,47.24 115.52,48.26 IC5.16 | JP1.6 142.65,48.26 141.53,47.14 129.03,47.14 127,49.17 MOSI.1
DISCK  (via drill 0.51)
  Top 0.203: JP1.8 143.56,45.72 145.09,44.2 145.09,38 143.66,36.58 121.82,36.58 120.29,38.1 IC5.12 115.32,38.1 111.76,41.66 107.29,41.66 105.56,43.38 v105.36,43.38
  Bottom 0.203: v105.36,43.38 99.16,43.38 98.55,43.99 98.55,45.52 97.74,46.33 97.74,49.48 91.54,55.68 80.57,55.68 79.15,57.1 73.66,57.1 IC3.12
DO_RESET  (via drill 0.51)
  Top 0.203: v130.05,69.29 130.56,69.29 v131.57,70.31
  Bottom 0.203: IC5.5 108.31,48.26 114.91,54.86 116.74,54.86 117.45,55.58 117.45,57.4 125.58,65.53 126.19,65.53 127.2,66.55 127.2,68.48 128.02,69.29 v130.05,69.29 | v131.57,70.31 135.33,70.31 140.92,75.89 140.92,76.2 JP2.7
DO_WD_LATCH
  Bottom 0.203: IC5.9 110.85,38.1 114.4,34.54 116.74,34.54 118.26,36.07 118.26,44.2 117.86,44.6 117.86,57.2 125.78,65.13 133.4,65.13 134.82,66.55 134.82,69.19 140.72,75.08 142.34,75.08 143.46,76.2 JP2.8
DOMOSI  (via drill 0.51)
  Top 0.203: IC4.13 50.8,54.97 55.78,59.94 55.78,63.5 v56.19,63.91 | v72.44,97.94 v70,95.5 | IC5.18 115.62,53.34 115.62,53.75 122.12,60.25 122.12,60.86 122.73,61.47 131.27,61.47 132.28,60.45 132.28,58.52 138.58,52.22 141.53,52.22 142.34,53.03 142.34,61.37 147.83,66.85 147.83,77.01 143.56,81.28 JP2.4
  Bottom 0.203: v56.19,63.91 56.19,72.34 57.71,73.86 59.54,73.86 68.07,82.4 68.07,91.03 70,92.96 v70,95.5 | v72.44,97.94 73.05,97.94 73.25,98.15 124.97,98.15 140.72,82.4 142.34,82.4 143.46,81.28 JP2.4
DOSCK  (via drill 0.51)
  Top 0.203: v48.67,52.73 48.67,54.97 50.8,57.1 IC4.12 | v145.9,42.57 145.9,38.2 143.87,36.17 119.08,36.17 117.86,37.39 117.04,37.39 116.74,37.08 111.15,37.08 108.61,39.62 106.78,39.62 v105.77,40.64
  Bottom 0.203: IC5.14 110.13,43.18 108.61,41.66 105.77,41.66 | 105.77,41.66 102.31,41.66 101.5,40.84 97.54,40.84 93.78,44.6 90.93,44.6 89.41,46.13 89.41,47.45 88.8,48.06 80.37,48.06 79.25,46.94 72.14,46.94 68.07,51 49.68,51 48.67,52.02 v48.67,52.73 | JP2.5 141.83,78.74 143.26,77.32 144.07,77.32 145.49,75.89 145.49,42.98 v145.9,42.57 | 105.77,41.66 v105.77,40.64
GND
  pour Route2 (no thermals): 0,99.06 149.86,99.06 149.86,0 0,0
GP3A0
  Top 0.203: IC3.28 81.28,85.14 88.9,85.14 SW1.9
GP3A1
  Bottom 0.203: IC3.27 81.28,82.6 88.9,82.6 SW1.10
GP3A2
  Bottom 0.203: IC3.26 81.28,80.06 88.9,80.06 SW1.11
GP3A3
  Bottom 0.203: IC3.25 81.28,77.52 88.9,77.52 SW1.12
GP3A4
  Bottom 0.203: IC3.24 81.28,74.98 88.9,74.98 SW1.13
GP3A5
  Bottom 0.203: IC3.23 81.28,72.44 88.9,72.44 SW1.14
GP3A6
  Bottom 0.203: IC3.22 81.28,69.9 88.9,69.9 SW1.15
GP3A7
  Bottom 0.203: IC3.21 81.28,67.26 88.9,67.26 SW1.16
GP3B0
  Bottom 0.203: BANK1.7 74.98,85.14 73.66,85.14 IC3.1
GP3B1
  Bottom 0.203: BANK1.9 74.98,82.6 73.66,82.6 IC3.2
GP3B2
  Bottom 0.203: IC3.3 73.66,80.26 84.84,91.44 86.36,91.44 BANK1.11
GP3B3
  Bottom 0.203: IC3.4 73.66,77.52 74.07,77.52 80.57,84.02 82.4,84.02 90.12,91.75 90.12,92.66 BANK1.13
GP3B4
  Bottom 0.203: IC3.5 73.66,75.29 71.93,77.01 71.93,77.93 72.95,78.94 74.78,78.94 79.55,83.72 79.55,85.55 85.04,91.03 87.78,91.03 88.9,92.15 88.9,93.27 89.61,93.98 91.44,93.98 BANK1.15
GP3B5
  Bottom 0.203: IC3.6 73.66,72.75 79.55,78.64 79.55,80.47 80.47,81.38 90.12,81.38 94.18,85.45 94.18,91.64 BANK1.17
GP3B6
  Bottom 0.203: IC3.7 73.66,70.21 79.55,76.1 79.55,77.93 80.47,78.84 90.12,78.84 94.59,83.31 94.59,89.51 BANK1.19
GP3B7
  Top 0.203: IC3.8 73.66,67.67 79.55,73.56 79.55,75.39 80.57,76.4 82.4,76.4 86.97,80.97 86.97,83.01 87.88,83.92 90.12,83.92 96.52,90.32 96.52,93.98 BANK1.20
GP4A0
  Top 0.203: IC4.21 58.42,67.67 60.15,69.39 60.15,70.81 68.78,79.45 69.19,79.45 69.29,79.35 70.1,79.35 71.93,81.18 71.93,85.55 77.83,91.44 78.74,91.44 BANK1.5
GP4A1
  Bottom 0.203: IC4.22 58.42,70.21 71.93,83.72 71.93,85.55 77.42,91.03 80.16,91.03 81.28,92.15 81.28,93.27 80.57,93.98 79.45,93.98 78.74,94.69 78.74,95.81 78.03,96.52 76.91,96.52 76.2,95.81 76.2,94.69 75.49,93.98 74.37,93.98 73.66,93.27 73.66,92.15 74.37,91.44 76.2,91.44 BANK1.3
GP4A2
  Bottom 0.203: BANK1.1 76.2,93.98 78.03,93.98 78.74,93.27 78.74,92.15 78.03,91.44 77.22,91.44 71.53,85.75 71.53,85.24 58.73,72.44 58.42,72.44 IC4.23
GP4A3
  Top 0.203: IC4.24 58.42,75.29 73.66,90.53 73.66,93.98 BANK1.2
GP4A4
  Bottom 0.203: IC4.25 58.42,77.83 67.67,87.07 67.67,91.24 68.58,92.15 68.58,93.98 BANK0.20
GP4A5
  Bottom 0.203: IC4.26 58.42,80.37 67.26,89.2 67.26,92.66 BANK0.19
GP4A6
  Bottom 0.203: IC4.27 58.42,82.91 64.72,89.2 64.72,92.66 BANK0.17
GP4A7
  Bottom 0.203: IC4.28 58.42,88.9 BANK0.15
GP4B0
  Bottom 0.203: IC4.1 50.8,95.81 49.68,96.93 46.13,96.93 BANK0.2
GP4B1
  Bottom 0.203: IC4.2 50.8,82.91 48.26,85.45 48.26,93.27 47.55,93.98 45.72,93.98 BANK0.1
GP4B2
  Bottom 0.203: IC4.3 50.8,80.37 47.04,84.12 47.04,92.66 BANK0.3
GP4B3
  Bottom 0.203: IC4.4 50.8,77.83 43.18,85.45 43.18,93.27 43.89,93.98 45.01,93.98 45.72,94.69 45.72,95.81 46.43,96.52 47.55,96.52 48.26,95.81 48.26,93.98 BANK0.5
GP4B4
  Bottom 0.203: IC4.5 50.8,75.29 52.53,77.01 52.53,92.25 BANK0.7
GP4B5
  Top 0.203: IC4.6 50.8,72.75 54.56,76.5 54.56,92.66 BANK0.9
GP4B6
  Top 0.203: IC4.7 50.8,70.21 52.83,72.24 52.83,74.17 56.29,77.62 56.29,91.85 BANK0.11
GP4B7
  Top 0.203: IC4.8 50.8,67.67 52.53,69.39 52.53,71.32 53.24,72.03 53.24,73.97 56.69,77.42 56.69,89.71 BANK0.13
GPIO28
  Bottom 0.203: BOB4.19 116.84,84.12 111.66,89.31 111.66,93.17 110.74,94.08 109.12,94.08 GPIO.4
GPIO33
  Bottom 0.203: BOB4.18 116.84,81.58 109.12,89.31 109.12,93.17 108.2,94.08 106.58,94.08 GPIO.2
GPIO34
  Bottom 0.203: BOB4.17 116.84,79.05 118.67,80.87 118.67,87.99 114.2,92.46 114.2,93.17 113.28,94.08 112.57,94.08 111.66,95 111.66,95.81 111.05,96.42 104.95,96.42 104.24,95.71 104.24,93.88 GPIO.1
GPIO39
  Bottom 0.203: BOB4.16 116.84,76.5 108,85.34 108,92.66 GPIO.3
GPIO40
  Top 0.203: BOB4.15 116.84,73.97 110.54,80.26 110.54,92.66 GPIO.5
GPIO41
  Top 0.203: BOB4.14 116.84,71.42 118.67,73.25 118.67,87.07 GPIO.7
GPIO42
  Top 0.203: BOB4.13 116.84,68.89 119.08,71.12 119.08,89.2 GPIO.9
GPIO55
  Top 0.203: BOB4.12 116.84,66.34 118.57,68.07 118.57,70 119.48,70.92 119.48,91.34 GPIO.10
HRTBT
  Top 0.203: U$1.2 28.85,10.16 30.18,11.48 35.66,11.48 36.17,11.99 R7.P$2
I2CRESET
  Bottom 0.203: BOB3.5 104.14,20.62 109.22,25.7 Q4.1
INTA3
  Bottom 0.203: BOB1.15 98.15,46.63 98.15,53.65 94.28,57.51 92.46,57.51 85.24,64.72 81.28,64.72 IC3.20
INTA4
  Top 0.203: BOB1.17 100.28,49.58 93.47,49.58 92.05,51 72.54,51 65.23,58.32 65.23,59.23 59.74,64.72 58.42,64.72 IC4.20
IRQ  (via drill 0.51)
  Top 0.203: v25.3,40.44 26.62,41.76 28.14,41.76 28.85,42.47 58.12,42.47 59.94,44.3 67.16,44.3 68.99,46.13 85.14,46.13 85.95,46.94 87.58,46.94 BOB1.5 | v22.05,41.76 18.9,41.76 U$1.53
  Bottom 0.203: v25.3,40.44 23.37,40.44 v22.05,41.76
IRQ5V
  Top 0.203: R16.P$2 104.14,46.94 104.24,46.84 118.06,46.84 119.48,45.41 119.48,45.01 119.89,44.6 120.5,44.6 IRQ.1 121.92,43.28 127.81,43.28 129.34,41.76 142.34,41.76 143.46,40.64 JP1.12
  Bottom 0.203: BOB1.16 100.38,46.94 101.4,46.94 103.83,44.5 104.65,44.5 105.05,44.91 105.05,46.02 104.14,46.94 R16.P$2 | JP1.12 143.56,40.64 143.56,41.55 145.09,43.08 145.09,69.6 141.02,73.66 JP2.9
J2_38
  Bottom 0.203: U$1.47 14.12,54.76 12.5,54.76 7.01,49.28 7.01,35.36 1.42,29.77 1.42,8.84 2.54,7.72 2.74,7.72 9.86,0.61 56.49,0.61 62.08,6.2 62.08,12.29 62.99,13.21 75.08,13.21 80.06,18.19 80.06,29.16 83.92,33.02 83.92,37.9 87.58,41.55 87.58,41.86 BOB1.7
J2_38_5
  Top 0.203: 137.21,56.13 140,53.34 JP1.1 | 137.21,56.13 134.82,58.52 134.82,60.45 133.4,61.87 116.74,61.87 109.73,54.86 107.29,54.86 106.17,53.75 106.17,53.14 101.5,48.46 97.43,48.46 95.2,46.23 95.2,45.21 98.45,41.96 100.28,41.96 BOB1.14 | 137.21,56.13 139.5,58.42 139.5,60.45 146.3,67.26 146.61,67.26 J238.1
  Bottom 0.203: JP2.6 143.56,78.74 143.56,78.44 146.61,75.39 146.61,67.36 J238.1
MISO0  (via drill 0.51)
  Top 0.203: v3.96,29.87 3.15,29.06 2.44,29.06 1.83,28.45 1.83,16.05 2.64,15.24 JP3.4
  Bottom 0.203: U$1.12 20.62,35.56 14.43,41.76 14.43,43.08 13.11,44.4 9.75,44.4 7.42,42.06 7.42,33.83 3.96,30.38 v3.96,29.87
MISO2
  Bottom 0.203: U$1.45 21.44,57 28.14,57 29.57,58.42 63.6,58.42 64.01,58.01 64.01,56.19 67.06,53.14 82.4,53.14 83.41,52.12 87.58,52.12 BOB1.3
MISO5
  Top 0.203: BOB1.18 100.28,52.02 89.92,52.02 88.8,53.14 74.68,53.14 73.66,52.12 IC3.14
  Bottom 0.203: IC4.14 50.8,52.12 56.19,52.12 57.2,53.14 66.45,53.14 67.46,52.12 73.66,52.12 IC3.14 | MISO.1 121.92,60.66 122.73,61.47 136.35,61.47 136.96,60.86 136.96,58.93 137.97,57.91 138.07,57.91 142.14,53.85 142.14,53.03 142.95,52.22 143.76,52.22 144.68,51.31 144.68,45.21 143.56,44.09 143.56,43.18 JP1.10 143.46,43.18 142.34,42.06 142.34,40.13 142.95,39.52 144.07,39.52 147.93,43.38 147.93,76 144.07,79.86 143.26,79.86 141.83,81.28 JP2.3 131.67,81.28 129.24,83.72 123.95,83.72 123.34,83.11 123.34,80.47 118.06,75.18 115.82,75.18 105.97,65.33 105.97,58.62 102.82,55.47 102.82,54.86 100.38,52.43 100.38,52.12 BOB1.18
MOSI0
  Bottom 0.203: U$1.11 27.94,32.11 21.84,26.01 21.84,21.54 21.44,21.13 21.44,19.81 20.52,18.9 11.28,18.9 JP3.5
MOSI2  (via drill 0.51)
  Top 0.203: U$1.44 20.32,54.25 21.84,55.78 v21.84,61.16 | v22.35,69.6 23.57,69.6 v24.18,70.21 | v104.95,58.83 107.9,55.88 IC5.2
  Bottom 0.203: IC5.4 108,50.8 108,51.21 109.73,52.93 109.73,54.15 108,55.88 IC5.2 | v21.84,61.16 21.84,69.09 v22.35,69.6 | v24.18,70.21 38.81,70.21 45.62,63.4 55.47,63.4 55.78,63.09 57.1,63.09 57.71,63.7 63.09,63.7 67.77,68.38 78.03,68.38 80.16,66.24 84.94,66.24 92.35,58.83 v104.95,58.83
N$2
  Bottom 0.203: D3.A 2.54,55.88 R6.P$1
N$3
  Bottom 0.203: C3.2@1 C3.2@2 67.36,33.02 68.58,31.8 71.12,31.8 76.2,26.72 TA8030S.1
N$4
  Bottom 0.203: TA8030S.2 73.66,26.62 75.59,24.69 76.71,24.69 78.74,26.72 R1.P$1 _.E 76.2,33.02 C6.1
N$5  (via drill 0.51)
  Top 0.203: BOB2.11 v100.99,18.39
  Bottom 0.203: BOB3.3 100.38,21.64 97.84,21.64 BOB2.11 | v100.99,18.39 100.99,8.53 102.92,6.6 108.61,6.6 111.15,4.06 116.23,4.06 117.35,2.95 117.35,2.34 118.16,1.52 127.31,1.52 131.57,5.79 132.69,5.79 134.62,3.86 I2C3.2
N$6  (via drill 0.51)
  Top 0.203: D1.A 64.72,38.1 64.11,38.71 62.69,38.71 62.08,38.1 D2.K v56.9,34.04
  Bottom 0.203: Q1.1 74.98,44.4 74.98,42.06 72.34,39.42 66.14,39.42 64.82,38.1 D1.A | v56.9,34.04 52.12,29.26 47.04,29.26 K0.1
N$9
  Top 0.203: D2.A R5.P$1
N$11
  Top 0.203: R4.P$1 91.44,19.81 89.41,21.84 89.41,28.04 78.74,38.71 R3.P$2
  Bottom 0.203: R3.P$2 74.88,36.78 64.31,36.78 63.5,37.59 63.5,38.61 64.31,39.42 64.72,39.42 67.77,42.47 73.66,42.47 Q1.2
N$12
  Bottom 0.203: Q3.2 92.76,23.57 92.76,24.79 97.74,29.77 R12.P$1
N$13  (via drill 0.51)
  Top 0.203: v97.74,38.1 97.74,38.81 94.69,41.86 R13.P$1
  Bottom 0.203: v97.74,38.1 97.74,37.19 99.16,35.76 101.09,35.76 106.98,29.87 110.44,29.87 Q4.2
N$14
  Bottom 2.184: WD.2 54.61,8.89 K0.4
N$15
  Top 2.184: K0.3 57.15,11.43 WD.3
N$16
  Bottom 0.203: BOB3.4 101.75,20.47 | 101.75,20.47 100.38,19.1 97.84,19.1 BOB2.10 | 101.75,20.47 102.92,19.3 112.78,19.3 115.32,21.84 120.6,21.84 121.11,22.35 121.11,23.67 127.81,30.38 131.27,30.38 145.09,16.56 145.09,11.38 143.97,10.26 143.66,10.26 138.58,5.18 138.58,2.74 137.67,1.83 134.01,1.83 132.08,3.76 I2C3.1
N$17
  Bottom 0.203: 91.44,28.55 91.44,30.48 94.59,33.63 94.59,34.24 R13.P$2 | 91.44,28.55 Q3.1 | R14.P$2 91.44,32.92 88.9,30.38 88.9,29.26 89.61,28.55 91.44,28.55
N$23
  Bottom 0.508: PWM.1 ULN2308.18
N$24
  Bottom 0.508: PWM.3 ULN2308.17
N$25
  Bottom 0.508: PWM.5 ULN2308.16
N$26
  Bottom 0.508: PWM.7 ULN2308.15
N$27
  Bottom 0.508: PWM.9 ULN2308.14
N$28
  Bottom 0.508: PWM.11 ULN2308.13
N$29
  Bottom 0.508: PWM.13 ULN2308.12
N$30
  Bottom 0.508: PWM.15 ULN2308.11
N$32
  Bottom 0.203: BOB5.2 35.56,82.09 28.65,89 26.52,89 25.5,90.02 25.5,90.83 24.69,91.64 22.86,91.64 21.54,90.32 DB9M.8
N$33
  Bottom 0.203: BOB5.4 30.48,83.62 26.92,87.17 26.92,87.99 24.69,90.22 24.28,90.22 DB9M.7
N$34
  Bottom 0.203: BOB5.1 38.1,79.96 35.76,77.62 27.84,77.62 26.52,78.94 26.52,83.82 DB9M.3
N$35
  Bottom 0.203: BOB5.3 33.02,79.96 31.09,78.03 29.97,78.03 29.16,78.84 29.16,84.02 25.7,87.48 DB9M.2
N$36
  Top 0.203: Q2.1 34.85,24.08 34.34,24.08 33.43,23.16 32.51,23.16 32,23.67 32,28.75 34.85,31.6 34.85,34.24 LED.K
N$37
  Bottom 0.203: R7.P$1 36.17,19.71 36.17,26.01 Q2.2
N$38
  Bottom 0.203: LED.A 37.49,34.34 41.86,34.34 R9.P$1
N$39
  Top 0.203: D4.P$1 85.04,61.27 85.04,62.69 85.55,63.2 89.92,63.2 91.44,61.67 R15.P$2
N$41
  Bottom 0.203: U$1.+5V 24.89,8.84 25.09,8.84 27.74,6.2 33.22,6.2 35.56,3.86 USB.1
N$42
  Top 0.203: U$1.D+ 24.89,13.92 24.89,13.01 26.82,11.07 26.82,9.65 27.64,8.84 33.12,8.84 38.1,3.86 USB.2
N$43
  Bottom 0.203: USB.3 40.64,6.3 36.78,10.16 36.27,10.16 35.05,11.38 24.89,11.38 U$1.D-
N$46
  Bottom 0.203: U$1.DE 19.41,20.32 18.09,21.64 5.08,21.64 3.86,22.86 DEBUG.2
N$47
  Bottom 0.203: U$1.DC 19.41,22.86 18.09,24.18 5.08,24.18 3.86,25.4 DEBUG.3
N$48
  Bottom 0.203: U$1.DD 20.32,27.03 13.11,34.24 9.75,34.24 8.33,32.82 8.33,32.31 3.96,27.94 DEBUG.4
NC
  Top 2.184: WD.1 50.8,5.08 50.8,16.51 52.96,18.67 K0.2
PROGRAM
  Top 0.203: SJ1.2 11.58,50.29 12.5,49.38 16.66,49.38 U$1.PROGRAM
PWM7
  Top 0.203: U$1.7 28.55,22.86 29.77,21.64 45.62,21.64 46.53,22.55 59.64,22.55 63.09,19.1 63.5,19.1 ULN2308.8
PWM21  (via drill 0.51)
  Top 0.203: v25.6,4.78 25.6,2.74 26.92,1.42 40.74,1.42 41.76,2.44 41.76,4.88 48.56,11.68 48.56,16.36 52.43,20.22 55.27,20.22 58.22,17.27 79.15,17.27 80.87,19 81.28,19 ULN2308.1
  Bottom 0.203: v25.6,4.78 24.99,4.78 15.65,14.12 13.82,14.12 U$1.21
PWM22
  Bottom 0.203: U$1.22 13.82,11.58 17.58,11.58 25.2,3.96 28.14,3.96 30.28,1.83 41.15,1.83 41.76,2.44 41.76,13.41 46.43,18.09 47.55,18.09 49.99,15.65 74.98,15.65 78.33,19 78.74,19 ULN2308.2
PWM23  (via drill 0.51)
  Top 0.203: v40.95,7.21 40.95,6.6 39.22,4.88 39.22,2.44 38.61,1.83 30.28,1.83 28.45,3.66 26.92,3.66 v26.42,3.15
  Bottom 0.203: ULN2308.3 76.2,18.8 73.46,16.05 50.19,16.05 47.75,18.49 46.23,18.49 41.25,13.51 41.25,7.52 v40.95,7.21 | v26.42,3.15 25.4,3.15 20.52,8.03 14.83,8.03 U$1.23
PWM29
  Bottom 0.203: U$1.29 25.7,53.34 22.05,49.68 20.12,49.68 19.2,48.77 19.2,48.06 18.29,47.14 17.58,47.14 16.66,46.23 16.66,42.67 17.27,42.06 20.52,42.06 25.6,36.98 28.14,36.98 29.06,36.07 29.06,35.36 30.07,34.34 31.09,34.34 33.02,32.41 33.02,31.8 33.63,31.19 39.93,31.19 54.25,16.87 71.12,16.87 73.25,19 73.66,19 ULN2308.4
PWM30
  Bottom 0.203: U$1.30 29.26,54.56 39.83,54.56 57.61,36.78 61.37,36.78 64.72,33.43 64.72,25.5 71.12,19.1 ULN2308.5
PWM35  (via drill 0.51)
  Top 0.203: v32.21,32 v34.04,32 | v13.61,41.86 6.81,41.86 v6.2,42.47
  Bottom 0.203: v34.04,32 39.73,32 44.5,27.23 48.26,27.23 58.22,17.27 66.45,17.27 68.17,19 68.58,19 ULN2308.6 | v32.21,32 31.09,32 30.89,31.8 30.07,31.8 29.06,32.82 29.06,33.53 28.14,34.44 21.03,34.44 v13.61,41.86 | v6.2,42.47 6.2,42.88 6.6,43.28 6.6,49.78 U$1.35
PWM36  (via drill 0.51)
  Top 0.203: v23.67,42.57 23.67,43.99 20.52,47.14 19.81,47.14 18.9,48.06 18.9,48.77 17.98,49.68 17.27,49.68 v15.54,51.41
  Bottom 0.203: v23.67,42.57 24.38,42.57 27.43,39.52 28.14,39.52 31.7,35.97 31.7,35.66 34.34,33.02 39.32,33.02 44.7,27.64 57.1,27.64 65.63,19.1 66.04,19.1 ULN2308.7 | v15.54,51.41 15.14,51.82 15.14,51.92 13.72,53.34 U$1.36
RESET  (via drill 0.51)
  Top 0.203: U$1.51 18.69,45.72 20.12,44.3 21.23,44.3 v21.84,43.69 | v46.43,41.25 76.91,41.25 79.05,43.38 89.1,43.38 89.15,43.43 | C8.1 89.15,43.43 | 89.15,43.43 90.12,42.47 90.12,29.87 R12.P$2 | v117.45,36.58 111.76,36.58 v111.45,36.27 | IC4.18 58.42,59.33 v65.43,52.32
  Bottom 0.203: IC4.18 58.42,59.74 64.72,59.74 65.73,60.76 80.26,60.76 81.28,59.74 IC3.18 | 115.62,45.72 115.62,46.13 117.35,47.85 117.35,49.07 115.62,50.8 IC5.17 | v21.84,43.69 22.86,43.69 22.96,43.79 25.7,43.79 27.74,41.76 45.92,41.76 v46.43,41.25 | 115.62,45.72 115.82,45.72 117.75,43.79 117.75,36.88 v117.45,36.58 | v111.45,36.27 109.42,36.27 108.61,37.08 102.31,37.08 101.09,38.3 98.75,38.3 98.15,38.91 97.33,38.91 92.76,34.34 92.76,32.41 90.22,29.87 R12.P$2 | 115.62,45.72 IC5.15 | v65.43,52.32 66.65,52.32 67.56,51.41 72.14,51.41 73.97,49.58 85.34,49.58 86.46,48.46 89,48.46 89.92,47.55 89.92,47.14 91.34,45.72 C8.1
RESETWD
  Top 0.203: R11.P$1 98.86,43.38 101.09,43.38 102.11,42.37 102.11,39.22 107.9,33.43 107.9,17.78 IC2.1
  Bottom 0.203: IC2.1 112.98,17.78 115.52,15.24 IC2.13 | R15.P$1 C8.2@2 C8.2@1 93.98,45.72 R11.P$1
RST1  (via drill 0.51)
  Top 0.203: R2.P$1 81.28,27.94 78.23,27.94 77.52,28.65 73.05,28.65 71.12,26.72 TA8030S.3 | v95.61,18.59 96.22,17.98 98.55,17.98 102.31,14.22 104.85,14.22 105.87,13.21 105.87,12.6 107.9,10.57 107.9,10.16 IC2.4
  Bottom 0.203: IC2.10 110.54,7.62 108,10.16 IC2.4 | v95.61,18.59 93.07,18.59 91.34,20.32 90.93,20.32 89.41,21.84 89.41,24.59 84.84,29.16 82.6,29.16 R2.P$1
RST/BOOT
  Top 0.203: JP3.16 SJ1.1
RTS4  (via drill 0.51)
  Top 0.203: U$1.26 27.94,46.63 26.52,48.06 26.52,48.77 23.06,52.22 19.81,52.22 18.9,53.14 18.9,53.85 17.98,54.76 17.27,54.76 v15.04,57
  Bottom 0.203: v15.04,57 15.04,61.06 4.88,71.22 2.54,71.22 1.42,72.34 1.42,80.67 3.25,82.5 3.76,82.5 FTDI.6 3.86,82.5 22.86,82.5 23.98,81.38 23.98,78.64 23.37,78.03 22.25,78.03 20.32,79.96 BOB5.8
RX1  (via drill 0.51)
  Top 0.203: U$1.0 27.74,5.08 25.6,7.21 18.59,7.21 v16.97,8.84
  Bottom 0.203: v16.97,8.84 14.94,8.84 13.82,9.96 13.82,10.67 12.9,11.58 11.28,11.58 JP3.3
RX4
  Bottom 0.203: U$1.31 27.94,58.73 24.08,62.59 24.08,69.09 17.78,75.39 17.78,78.03 | BOB5.9 17.78,78.03 | 17.78,78.03 14.73,78.03 12.8,79.96 3.86,79.96 FTDI.5
SC0
  Bottom 0.203: BOB3.10 104.14,7.92 106.17,9.96 106.17,10.57 106.88,11.28 125.58,11.28 I2C3_0-1.3
SC1
  Top 0.203: BOB3.12 105.77,2.54 107.29,4.06 109.83,4.06 114.91,9.14 124.36,9.14 128.02,12.8 129.64,12.8 I2C3_0-1.4
SC2
  Top 0.203: BOB3.14 122.63,8.33 128.32,8.33 129.84,9.86 136.85,9.86 I2C3_2-3.3
SC3
  Bottom 0.203: BOB3.16 134.72,10.16 137.36,12.8 142.34,12.8 I2C3_2-3.4
SC4
  Bottom 0.203: BOB3.18 119.38,15.54 127.1,23.27 127.1,25.5 I2C3_4-5.3
SC5
  Top 0.203: BOB3.20 122.83,20.32 128.02,25.5 129.64,25.5 I2C3_4-5.4
SC6
  Bottom 0.203: BOB3.22 122.22,25.4 127.61,30.79 136.85,30.79 I2C3_6-7.3
SC7
  Bottom 0.203: BOB3.24 126.69,30.48 127.41,31.19 137.36,31.19 140.72,27.84 142.34,27.84 I2C3_6-7.4
SCK0
  Top 0.203: U$1.13 11.79,35.56 10.46,34.24 9.75,34.24 8.94,33.43 8.94,21.54 JP3.6
SCK2  (via drill 0.51)
  Top 0.203: v23.27,68.68 24.49,68.68 v24.89,69.09 | v104.24,45.31 107.49,45.31 107.9,45.72 IC5.6 108,45.72 109.02,44.7 116.74,44.7 117.04,45.01 v118.67,45.01
  Bottom 0.203: IC5.8 113.39,40.64 114.91,42.16 116.74,42.16 117.35,42.77 117.35,43.59 116.23,44.7 109.02,44.7 108,45.72 IC5.6 | U$1.46 23.27,61.37 v23.27,68.68 | v24.89,69.09 24.89,62.38 27.74,59.54 28.45,59.54 28.75,59.23 48.16,59.23 49.68,60.76 55.88,60.76 56.19,60.45 57,60.45 57.71,61.16 61.16,61.16 67.16,67.16 71.63,67.16 72.95,65.84 84.73,65.84 92.66,57.91 94.49,57.91 98.55,53.85 98.55,49.07 99.57,48.06 101.5,48.06 102.82,46.74 102.82,46.53 104.04,45.31 v104.24,45.31 | v118.67,45.01 SPICLK.1
SCL0
  Top 0.203: JP4.11 36.78,10.16 37.19,9.75 38.41,9.75 39.93,11.28 39.93,11.99 R8.P$1
  Bottom 0.203: U$1.19 11.79,20.32 10.46,19 9.75,19 8.94,18.19 8.94,17.37 9.86,16.46 18.29,16.46 24.69,10.06 26.42,10.06 27.43,9.04 29.36,9.04 JP4.11
SCL1  (via drill 0.51)
  Top 0.203: v58.12,1.02 20.93,1.02 15.54,6.4 8.74,6.4 4.88,10.26 2.54,10.26 0.61,12.19 0.61,41.86 9.04,50.29 9.04,51 9.25,51.21 12.29,51.21 U$1.37
  Bottom 0.203: v58.12,1.02 62.08,4.98 81.58,4.98 82.5,5.89 82.5,8.53 87.58,13.61 87.58,13.92 BOB2.5
SCL1_5V
  Bottom 0.203: BOB2.8 97.74,13.92 97.74,13.61 93.17,9.04 93.17,5.49 92.56,4.88 92.56,2.44 91.95,1.83 90.83,1.83 88.9,3.76 I2C1.1
SCL3  (via drill 0.51)
  Top 0.203: v77.72,20.83 77.83,20.93 84.94,20.93 86.77,19.1 87.58,19.1 BOB2.3
  Bottom 0.203: v77.72,20.83 75.79,20.83 74.68,19.71 74.68,17.88 73.25,16.46 54.05,16.46 41.35,29.16 30.07,29.16 29.06,28.14 29.06,27.43 28.14,26.52 27.43,26.52 21.84,20.93 21.84,17.68 20.83,16.66 18.9,16.66 U$1.57
SD0
  Bottom 0.203: BOB3.9 105.16,10.16 106.68,11.68 123.44,11.68 I2C3_0-1.1
SD1
  Top 0.203: BOB3.11 105.77,5.08 107.29,6.6 109.83,6.6 114.91,11.68 124.36,11.68 128.02,15.34 129.64,15.34 I2C3_0-1.2
SD2
  Bottom 0.203: BOB3.13 127.71,2.54 135.43,10.26 141.43,10.26 142.34,11.18 142.34,11.89 143.26,12.8 143.97,12.8 144.68,13.51 144.68,14.43 143.76,15.34 142.14,15.34 I2C3_2-3.1
SD3
  Top 0.203: BOB3.15 121.31,7.62 122.43,8.74 127.61,8.74 129.13,10.26 135.64,10.26 140.72,15.34 142.34,15.34 I2C3_2-3.2
SD4
  Bottom 0.203: BOB3.17 119.38,13.01 117.65,14.73 117.65,20.83 118.26,21.44 120.8,21.44 128.22,28.85 128.22,29.16 I2C3_4-5.1
SD5
  Bottom 0.203: BOB3.19 119.38,18.09 126.69,25.4 126.69,26.72 128.02,28.04 129.64,28.04 I2C3_4-5.2
SD6
  Bottom 0.203: BOB3.21 119.38,23.16 117.65,24.89 117.65,30.99 118.26,31.6 138.58,31.6 I2C3_6-7.1
SD7
  Top 0.203: BOB3.23 121.82,30.38 142.34,30.38 I2C3_6-7.2
SDA0
  Top 0.203: U$1.18 13.72,22.86 15.14,21.44 25.2,21.44 27.64,19 34.85,19 41.25,12.6 41.25,11.48 38.71,8.94 36.27,8.94 R10.P$1
  Bottom 0.203: JP4.12 34.95,7.62 36.17,8.84 R10.P$1
SDA1  (via drill 0.51)
  Top 0.203: v56.08,1.83 57.71,1.83 60.86,4.98 79.05,4.98 79.96,5.89 79.96,6.71 85.85,12.6 85.85,14.43 87.58,16.15 87.58,16.46 BOB2.4 | v2.74,29.87 2.74,30.48 v1.83,31.39 | v5.79,43.69 9.04,43.69 9.86,44.5 10.57,44.5 11.58,45.52 11.58,47.14 U$1.38
  Bottom 0.203: v56.08,1.83 44.3,1.83 43.48,1.02 20.93,1.02 15.44,6.5 12.19,6.5 11.38,7.32 11.38,8.03 10.46,8.94 8.74,8.94 4.88,12.8 2.54,12.8 1.83,13.51 1.83,28.96 v2.74,29.87 | v1.83,31.39 1.83,42.37 3.15,43.69 v5.79,43.69
SDA1_5V
  Bottom 0.203: I2C1.2 91.44,4.37 92.76,5.69 92.76,11.18 97.74,16.15 97.74,16.46 BOB2.9
SDA3  (via drill 0.51)
  Top 0.203: v46.02,23.27 59.54,23.27 61.16,21.64 87.58,21.64 BOB2.2 | v31.5,16.56 26.42,16.56 25.09,17.88 21.84,17.88 20.52,19.2 18.9,19.2 U$1.56
  Bottom 0.203: v46.02,23.27 41.55,23.27 34.85,16.56 v31.5,16.56
TX1
  Top 0.203: U$1.1 19.41,7.62 15.75,11.28 11.28,11.28 JP3.2
TX4
  Top 0.203: U$1.32 27.43,60.96 25.6,62.79 25.6,68.58 25.7,68.68 25.7,77.11 22.86,79.96 BOB5.7
  Bottom 0.203: FTDI.4 1.83,79.45 1.83,80.47 2.74,81.38 14.12,81.38 14.73,81.99 20.93,81.99 22.86,80.06 BOB5.7
VBAT
  Top 0.203: U$1.VBAT 25.4,48.06 23.06,45.72 23.06,45.21 24.49,43.79 24.49,39.93 27.74,36.68 29.36,36.68 JP4.1
VCC  (via drill 0.51)
  Top 0.508: BOB1.20 100.38,57.1 101.6,57.1 104.14,54.56 R16.P$1
  Bottom 0.508: v98.75,55.88 99.97,57.1 100.28,57.1 BOB1.20 | R14.P$1 91.44,41.96 90.02,41.96 88.8,43.18 86.46,43.18 82.6,39.32 82.6,36.88 R2.P$2
  pour Route15 (isolate 0.61, rank 3, no thermals): 0,99.06 149.86,99.06 149.86,0 0,0
WD_LATCH_3
  Top 0.203: U$1.54 26.62,34.24 30.79,34.24 35.97,39.42 75.69,39.42 78.23,41.96 79.25,41.96 81.79,39.42 87.58,39.42 BOB1.8
WD_LATCH_5
  Bottom 0.203: 113.79,39.42 114.3,39.42 115.52,40.64 IC5.13 | 113.79,39.42 100.38,39.42 BOB1.13 100.28,39.32 94.69,39.32 90.12,34.75 90.12,34.54 88.8,33.22 84.73,33.22 81.28,29.77 81.28,25.7 86.46,20.52 88.39,20.52 89,19.91 91.14,19.91 93.27,17.78 98.75,17.78 99.57,16.97 99.57,9.35 102.72,6.2 105.26,6.2 105.87,5.59 105.87,4.98 106.78,4.06 108.61,4.06 110.13,2.54 IC2.8 | 113.79,39.42 113.79,37.69 115.52,35.97 115.52,35.56 IC5.11
WD_RFSH
  Bottom 0.203: U$1.52 18.69,43.18 20.02,44.5 44.4,44.5 WDRFSH.1 54.05,38.1 59.13,33.02 C3.1
WDOUT
  Top 0.203: IC2.5 106.38,7.62 104.85,9.14 92.46,9.14 R4.P$2

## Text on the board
tPlace: 20 | 20 | 10 | 1 | 1 | 1 | +5V | gnd | TX4/Rx4 | RTS | BS0 | RxD | MISO | MOSI | TxD | SCK | J238 | Vcc | RST | WD | CTS | IRQ | Gnd | R2Out | R1Out | T2In | T1In | Gnd | Vcc | R2In | R1In | T2Out | T1Out | Gnd | CTS | RxD | RTS | TxD | Pwr | J238 | WD | vcc | BS1 | Gnd | BS2 | MOSI | 3.3v | BS3 | SCK | BS4 | MISO | 1 | G | Weensy 3.6 / Copyright 2017 / Plantation / Productions, Inc. / Rev 4 | BS5 | IRQ | 1 | BS6 | RST | 0 | SD4 | SD5 | SD6 | SD7 | SC4 | SC5 | SC6 | SC7 | 1 | Gnd | Gnd | Gnd | Gnd | A0- | SD0 | SD1 | SD2 | SD3 | A0+ | SC0 | SC1 | SC2 | SC3 | AR | Gnd | Gnd | Gnd | Gnd | AG | 1 | NC | COM | NO | SCL | SDA | +5V | Gnd | SCL | SDA | +5V | Gnd | 16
